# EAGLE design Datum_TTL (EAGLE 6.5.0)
dasdad

## Sheet 1 of 3: Tag
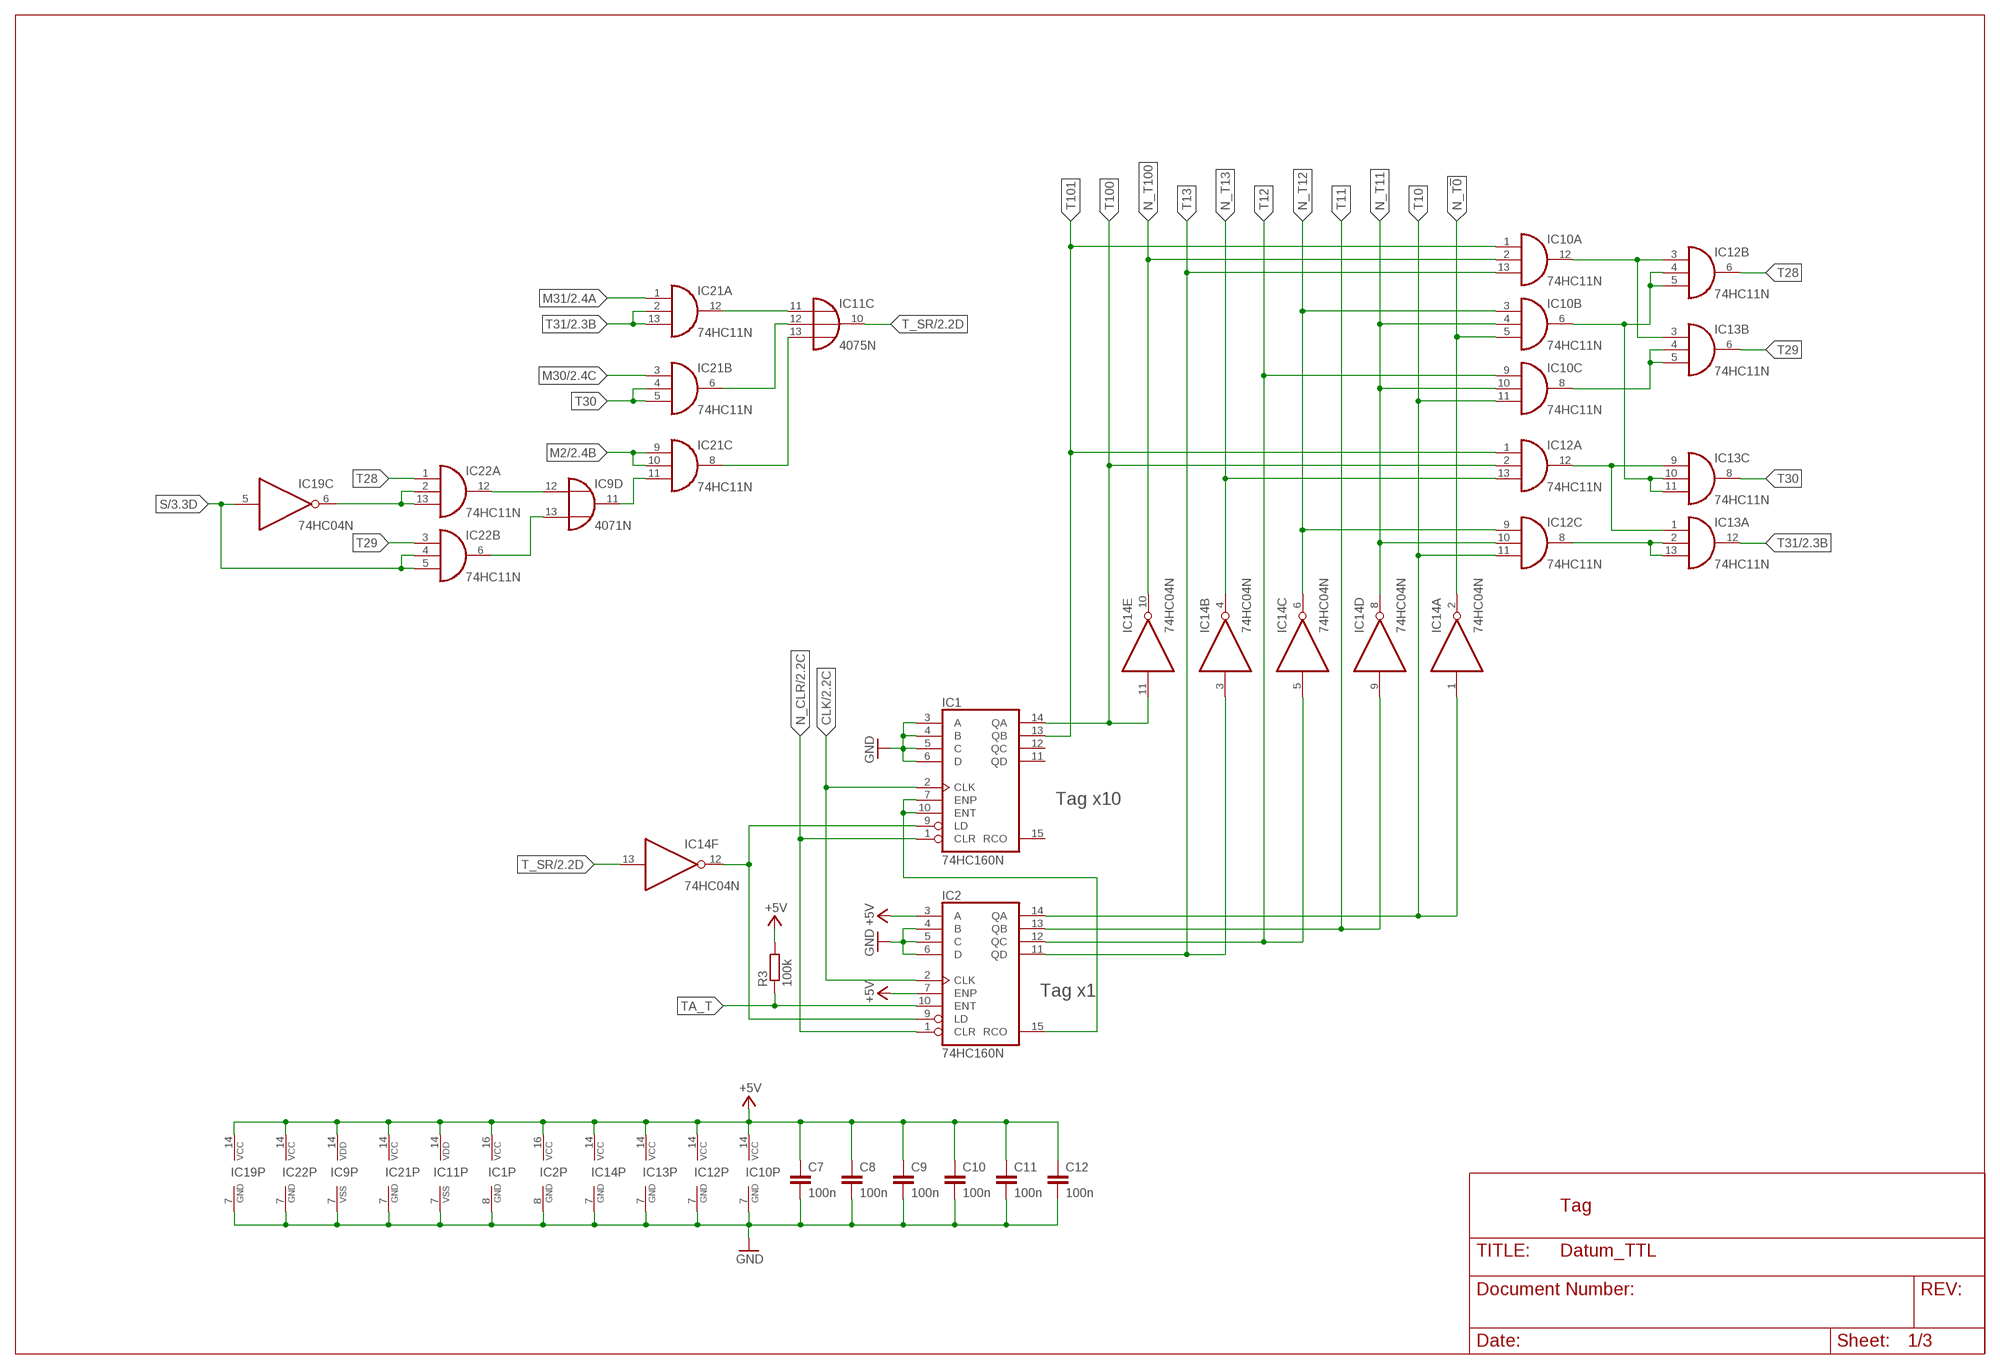
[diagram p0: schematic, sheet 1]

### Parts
C7  100n  C-EU025-024X044  [C025-024X044]
C8  100n  C-EU025-024X044  [C025-024X044]
C9  100n  C-EU025-024X044  [C025-024X044]
C10  100n  C-EU025-024X044  [C025-024X044]
C11  100n  C-EU025-024X044  [C025-024X044]
C12  100n  C-EU025-024X044  [C025-024X044]
IC1  74HC160N  [DIL16]
IC2  74HC160N  [DIL16]
IC9  4071N  [DIL14]
IC10  74HC11N  [DIL14]
IC11  4075N  [DIL14]
IC12  74HC11N  [DIL14]
IC13  74HC11N  [DIL14]
IC14  74HC04N  [DIL14]
IC19  74HC04N  [DIL14]
IC21  74HC11N  [DIL14]
IC22  74HC11N  [DIL14]
R3  100k  R-EU_0207/10  [0207/10]

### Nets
+5V: C7.1 C8.1 C9.1 C10.1 C11.1 C12.1 IC1.16(VCC) IC2.3(A) IC2.7(ENP) IC2.16(VCC) IC9.14(P:VDD) IC10.14(P:VCC) IC11.14(P:VDD) IC12.14(P:VCC) IC13.14(P:VCC) IC14.14(P:VCC) IC19.14(P:VCC) IC21.14(P:VCC) IC22.14(P:VCC) R3.2 ; also sheet 2,3
CLK: IC1.2(CLK) IC2.2(CLK) ; also sheet 2,3
GND: C7.2 C8.2 C9.2 C10.2 C11.2 C12.2 IC1.3(A) IC1.4(B) IC1.5(C) IC1.6(D) IC1.8(GND) IC2.4(B) IC2.5(C) IC2.6(D) IC2.8(GND) IC9.7(P:VSS) IC10.7(P:GND) IC11.7(P:VSS) IC12.7(P:GND) IC13.7(P:GND) IC14.7(P:GND) IC19.7(P:GND) IC21.7(P:GND) IC22.7(P:GND) ; also sheet 2,3
M2: IC21.9(C:I0) IC21.10(C:I1) ; also sheet 2
M30: IC21.3(B:I0) ; also sheet 2
M31: IC21.1(A:I0) ; also sheet 2
N$2: IC1.7(ENP) IC1.10(ENT) IC2.15(RCO)
N$21: IC10.12(A:O) IC12.3(B:I0) IC13.3(B:I0)
N$22: IC10.6(B:O) IC12.4(B:I1) IC12.5(B:I2) IC13.10(C:I1) IC13.11(C:I2)
N$23: IC12.8(C:O) IC13.2(A:I1) IC13.13(A:I2)
N$24: IC10.8(C:O) IC13.4(B:I1) IC13.5(B:I2)
N$25: IC12.12(A:O) IC13.1(A:I0) IC13.9(C:I0)
N$36: IC9.12(D:I0) IC22.12(A:O)
N$37: IC9.13(D:I1) IC22.6(B:O)
N$38: IC9.11(D:O) IC21.11(C:I2)
N$39: IC11.11(C:I0) IC21.12(A:O)
N$41: IC19.6(C:O) IC22.2(A:I1) IC22.13(A:I2)
N$42: IC11.12(C:I1) IC21.6(B:O)
N$43: IC11.13(C:I2) IC21.8(C:O)
N_CLR: IC1.1(CLR) IC2.1(CLR) ; also sheet 2,3
N_T11: IC10.4(B:I1) IC10.10(C:I1) IC12.10(C:I1) IC14.8(D:O)
N_T12: IC10.3(B:I0) IC12.9(C:I0) IC14.6(C:O)
N_T13: IC12.13(A:I2) IC14.4(B:O)
N_T100: IC10.2(A:I1) IC14.10(E:O)
N_T!0: IC10.5(B:I2) IC14.2(A:O)
N_T_SR: IC1.9(LD) IC2.9(LD) IC14.12(F:O)
S: IC19.5(C:I) IC22.4(B:I1) IC22.5(B:I2) ; also sheet 3
T10: IC2.14(QA) IC10.11(C:I2) IC12.11(C:I2) IC14.1(A:I) ; also sheet 3
T11: IC2.13(QB) IC14.9(D:I) ; also sheet 3
T12: IC2.12(QC) IC10.9(C:I0) IC14.5(C:I) ; also sheet 3
T13: IC2.11(QD) IC10.13(A:I2) IC14.3(B:I) ; also sheet 3
T28: IC12.6(B:O) IC22.1(A:I0)
T29: IC13.6(B:O) IC22.3(B:I0)
T30: IC13.8(C:O) IC21.4(B:I1) IC21.5(B:I2)
T31: IC13.12(A:O) IC21.2(A:I1) IC21.13(A:I2) ; also sheet 2
T100: IC1.14(QA) IC12.2(A:I1) IC14.11(E:I) ; also sheet 3
T101: IC1.13(QB) IC10.1(A:I0) IC12.1(A:I0) ; also sheet 3
T_SR: IC11.10(C:O) IC14.13(F:I) ; also sheet 2
TA_T: IC2.10(ENT) R3.1 ; also sheet 3
Unconnected: IC1.11(QD) IC1.12(QC) IC1.15(RCO)

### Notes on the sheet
- Tag x10
- Tag x1
- Tag

## Sheet 2 of 3: Monat
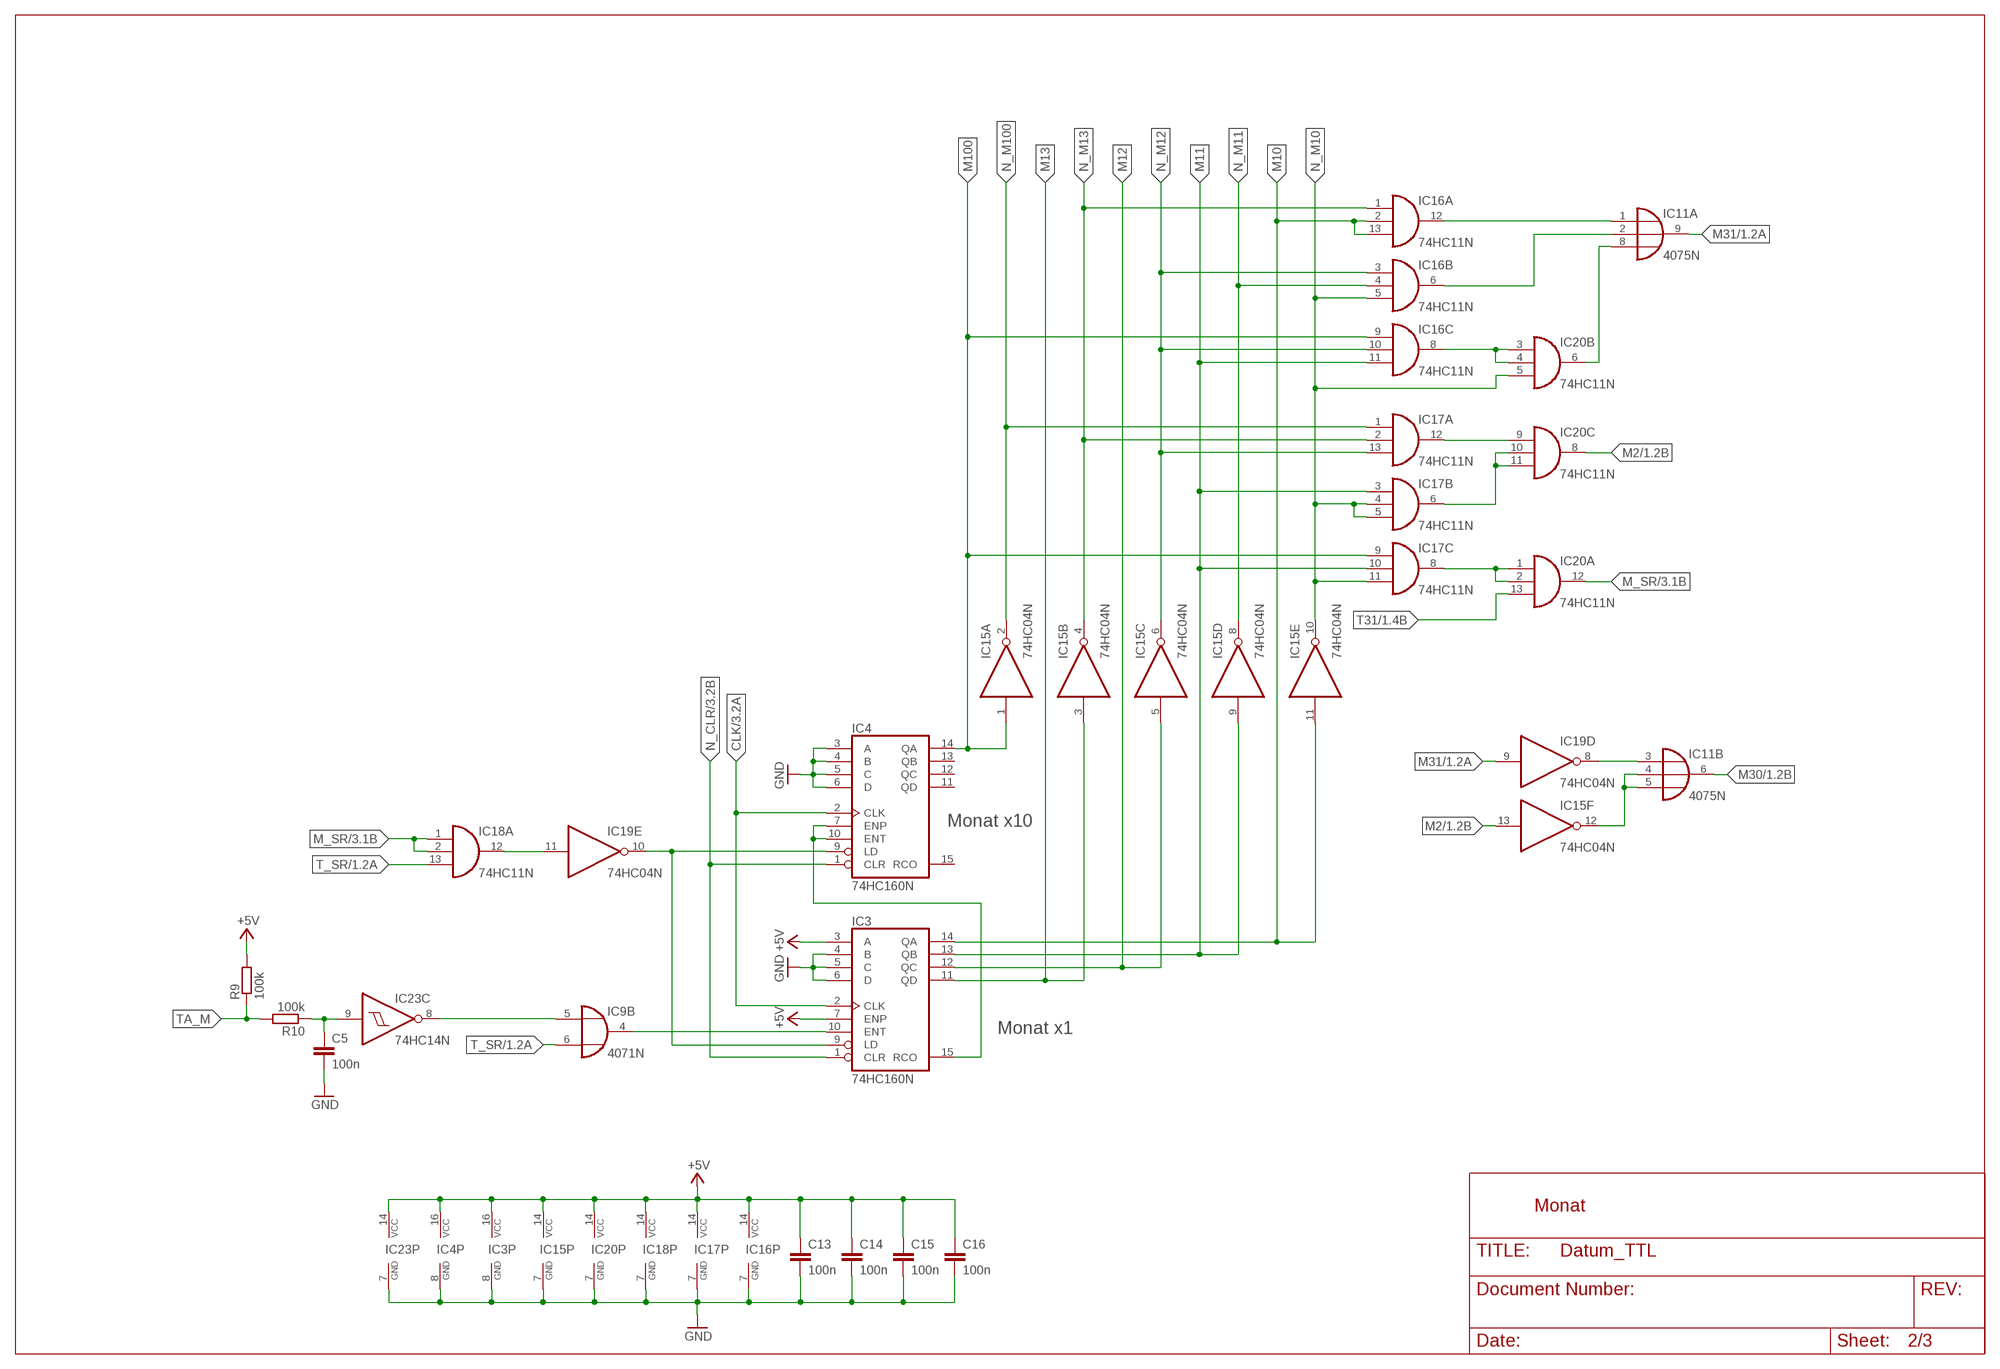
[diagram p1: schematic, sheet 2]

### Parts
C5  100n  C-EU025-024X044  [C025-024X044]
C13  100n  C-EU025-024X044  [C025-024X044]
C14  100n  C-EU025-024X044  [C025-024X044]
C15  100n  C-EU025-024X044  [C025-024X044]
C16  100n  C-EU025-024X044  [C025-024X044]
IC3  74HC160N  [DIL16]
IC4  74HC160N  [DIL16]
IC15  74HC04N  [DIL14]
IC16  74HC11N  [DIL14]
IC17  74HC11N  [DIL14]
IC18  74HC11N  [DIL14]
IC20  74HC11N  [DIL14]
IC23  74HC14N  [DIL14]
R9  100k  R-EU_0207/10  [0207/10]
R10  100k  R-EU_0207/10  [0207/10]

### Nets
+5V: C13.1 C14.1 C15.1 C16.1 IC3.3(A) IC3.7(ENP) IC3.16(VCC) IC4.16(VCC) IC15.14(P:VCC) IC16.14(P:VCC) IC17.14(P:VCC) IC18.14(P:VCC) IC20.14(P:VCC) IC23.14(P:VCC) R9.2 ; also sheet 1,3
CLK: IC3.2(CLK) IC4.2(CLK) ; also sheet 1,3
GND: C5.2 C13.2 C14.2 C15.2 C16.2 IC3.4(B) IC3.5(C) IC3.6(D) IC3.8(GND) IC4.3(A) IC4.4(B) IC4.5(C) IC4.6(D) IC4.8(GND) IC15.7(P:GND) IC16.7(P:GND) IC17.7(P:GND) IC18.7(P:GND) IC20.7(P:GND) IC23.7(P:GND) ; also sheet 1,3
M2: IC15.13(F:I) IC20.8(C:O) ; also sheet 1
M10: IC3.14(QA) IC15.11(E:I) IC16.2(A:I1) IC16.13(A:I2) ; also sheet 3
M11: IC3.13(QB) IC15.9(D:I) IC16.11(C:I2) IC17.3(B:I0) IC17.10(C:I1) ; also sheet 3
M12: IC3.12(QC) IC15.5(C:I) ; also sheet 3
M13: IC3.11(QD) IC15.3(B:I) ; also sheet 3
M30: IC11.6(B:O) ; also sheet 1
M31: IC11.9(A:O) IC19.9(D:I) ; also sheet 1
M100: IC4.14(QA) IC15.1(A:I) IC16.9(C:I0) IC17.9(C:I0) ; also sheet 3
M_SR: IC18.1(A:I0) IC18.2(A:I1) IC20.12(A:O) ; also sheet 3
N$3: IC9.5(B:I0) IC23.8(C:O)
N$4: IC18.12(A:O) IC19.11(E:I)
N$6: IC3.15(RCO) IC4.7(ENP) IC4.10(ENT)
N$7: IC3.10(ENT) IC9.4(B:O)
N$8: IC3.9(LD) IC4.9(LD) IC19.10(E:O)
N$14: IC17.8(C:O) IC20.1(A:I0) IC20.2(A:I1)
N$26: IC11.1(A:I0) IC16.12(A:O)
N$27: IC11.2(A:I1) IC16.6(B:O)
N$28: IC11.8(A:I2) IC20.6(B:O)
N$29: IC16.8(C:O) IC20.3(B:I0) IC20.4(B:I1)
N$30: IC17.12(A:O) IC20.9(C:I0)
N$31: IC17.6(B:O) IC20.10(C:I1) IC20.11(C:I2)
N$32: IC11.3(B:I0) IC19.8(D:O)
N$33: IC11.4(B:I1) IC11.5(B:I2) IC15.12(F:O)
N$77: C5.1 IC23.9(C:I) R10.1
N_CLR: IC3.1(CLR) IC4.1(CLR) ; also sheet 1,3
N_M10: IC15.10(E:O) IC16.5(B:I2) IC17.4(B:I1) IC17.5(B:I2) IC17.11(C:I2) IC20.5(B:I2)
N_M11: IC15.8(D:O) IC16.4(B:I1)
N_M12: IC15.6(C:O) IC16.3(B:I0) IC16.10(C:I1) IC17.13(A:I2)
N_M13: IC15.4(B:O) IC16.1(A:I0) IC17.2(A:I1)
N_M100: IC15.2(A:O) IC17.1(A:I0)
T31: IC20.13(A:I2) ; also sheet 1
T_SR: IC9.6(B:I1) IC18.13(A:I2) ; also sheet 1
TA_M: R9.1 R10.2 ; also sheet 3
Unconnected: IC4.11(QD) IC4.12(QC) IC4.13(QB) IC4.15(RCO)

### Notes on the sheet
- Monat x10
- Monat x1
- Monat

## Sheet 3 of 3: Jahr, Wochentag, IO
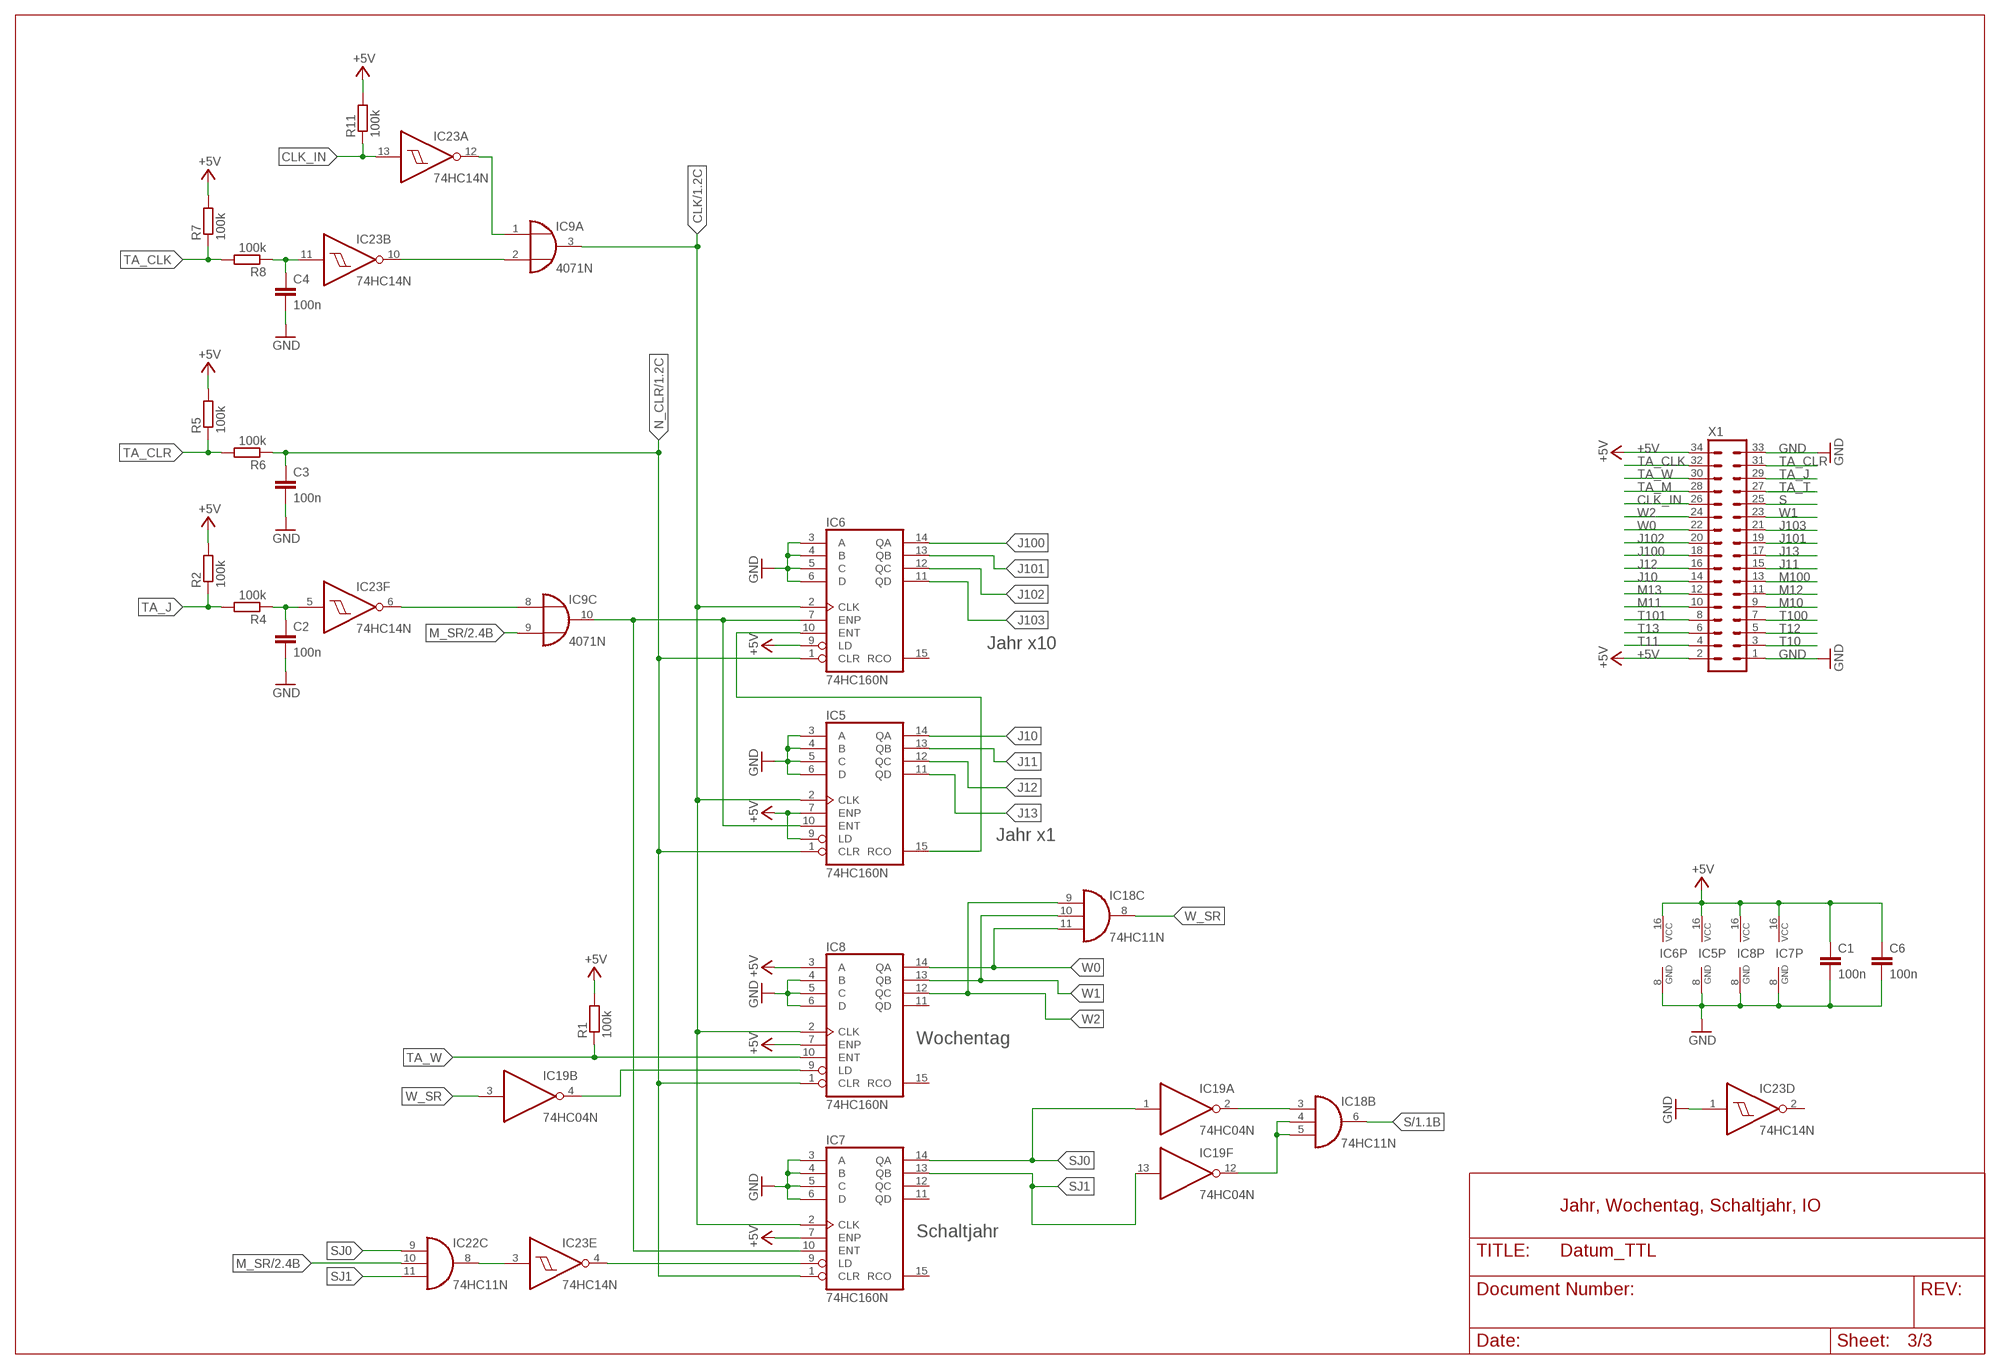
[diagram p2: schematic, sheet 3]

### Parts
C1  100n  C-EU025-024X044  [C025-024X044]
C2  100n  C-EU025-024X044  [C025-024X044]
C3  100n  C-EU025-024X044  [C025-024X044]
C4  100n  C-EU025-024X044  [C025-024X044]
C6  100n  C-EU025-024X044  [C025-024X044]
IC5  74HC160N  [DIL16]
IC6  74HC160N  [DIL16]
IC7  74HC160N  [DIL16]
IC8  74HC160N  [DIL16]
R1  100k  R-EU_0207/10  [0207/10]
R2  100k  R-EU_0207/10  [0207/10]
R4  100k  R-EU_0207/10  [0207/10]
R5  100k  R-EU_0207/10  [0207/10]
R6  100k  R-EU_0207/10  [0207/10]
R7  100k  R-EU_0207/10  [0207/10]
R8  100k  R-EU_0207/10  [0207/10]
R11  100k  R-EU_0207/10  [0207/10]
X1  ML34  [ML34]

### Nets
+5V: C1.1 C6.1 IC5.7(ENP) IC5.9(LD) IC5.16(VCC) IC6.9(LD) IC6.16(VCC) IC7.7(ENP) IC7.16(VCC) IC8.3(A) IC8.7(ENP) IC8.16(VCC) R1.2 R2.2 R5.2 R7.2 R11.2 X1.2 X1.34 ; also sheet 1,2
CLK: IC5.2(CLK) IC6.2(CLK) IC7.2(CLK) IC8.2(CLK) IC9.3(A:O) ; also sheet 1,2
CLK_IN: IC23.13(A:I) R11.1 X1.26
GND: C1.2 C2.2 C3.2 C4.2 C6.2 IC5.3(A) IC5.4(B) IC5.5(C) IC5.6(D) IC5.8(GND) IC6.3(A) IC6.4(B) IC6.5(C) IC6.6(D) IC6.8(GND) IC7.3(A) IC7.4(B) IC7.5(C) IC7.6(D) IC7.8(GND) IC8.4(B) IC8.5(C) IC8.6(D) IC8.8(GND) IC23.1(D:I) X1.1 X1.33 ; also sheet 1,2
J10: IC5.14(QA) X1.14
J11: IC5.13(QB) X1.15
J12: IC5.12(QC) X1.16
J13: IC5.11(QD) X1.17
J100: IC6.14(QA) X1.18
J101: IC6.13(QB) X1.19
J102: IC6.12(QC) X1.20
J103: IC6.11(QD) X1.21
M10: X1.9 ; also sheet 2
M11: X1.10 ; also sheet 2
M12: X1.11 ; also sheet 2
M13: X1.12 ; also sheet 2
M100: X1.13 ; also sheet 2
M_SR: IC9.9(C:I1) IC22.10(C:I1) ; also sheet 2
N$1: C2.1 IC23.5(F:I) R4.1
N$5: IC9.1(A:I0) IC23.12(A:O)
N$9: IC22.8(C:O) IC23.3(E:I)
N$10: IC5.15(RCO) IC6.10(ENT)
N$11: IC5.10(ENT) IC6.7(ENP) IC7.10(ENT) IC9.10(C:O)
N$13: IC7.9(LD) IC23.4(E:O)
N$15: IC9.8(C:I0) IC23.6(F:O)
N$16: IC8.9(LD) IC19.4(B:O)
N$17: IC9.2(A:I1) IC23.10(B:O)
N$19: C4.1 IC23.11(B:I) R8.1
N$34: IC18.3(B:I0) IC19.2(A:O)
N$35: IC18.4(B:I1) IC18.5(B:I2) IC19.12(F:O)
N_CLR: C3.1 IC5.1(CLR) IC6.1(CLR) IC7.1(CLR) IC8.1(CLR) R6.1 ; also sheet 1,2
S: IC18.6(B:O) X1.25 ; also sheet 1
SJ0: IC7.14(QA) IC19.1(A:I) IC22.9(C:I0)
SJ1: IC7.13(QB) IC19.13(F:I) IC22.11(C:I2)
T10: X1.3 ; also sheet 1
T11: X1.4 ; also sheet 1
T12: X1.5 ; also sheet 1
T13: X1.6 ; also sheet 1
T100: X1.7 ; also sheet 1
T101: X1.8 ; also sheet 1
TA_CLK: R7.1 R8.2 X1.32
TA_CLR: R5.1 R6.2 X1.31
TA_J: R2.1 R4.2 X1.29
TA_M: X1.28 ; also sheet 2
TA_T: X1.27 ; also sheet 1
TA_W: IC8.10(ENT) R1.1 X1.30
W0: IC8.14(QA) IC18.11(C:I2) X1.22
W1: IC8.13(QB) IC18.10(C:I1) X1.23
W2: IC8.12(QC) IC18.9(C:I0) X1.24
W_SR: IC18.8(C:O) IC19.3(B:I)
Unconnected: IC6.15(RCO) IC7.11(QD) IC7.12(QC) IC7.15(RCO) IC8.11(QD) IC8.15(RCO) IC23.2(D:O)

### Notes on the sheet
- Jahr x10
- Jahr x1
- Wochentag
- Jahr, Wochentag, Schaltjahr, IO
- Schaltjahr

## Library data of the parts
C1-C16 = rcl:C-EU: CAPACITOR, European symbol
IC1-IC8 = 74xx-eu:74*160: Synchronous 4-bit COUNTER
IC9 = 40xx:4071: Quad 2-input OR
IC10 IC12 IC13 IC16-IC18 IC20-IC22 = 74xx-eu:74*11: Triple 3-input AND gate
IC11 = 40xx:4075: Triple 3-input OR
IC14 IC15 IC19 = 74xx-eu:74*04: Hex INVERTER
IC23 = 74xx-eu:74*14: Hex schmitt trigger INVERTER
R1-R11 = rcl:R-EU_: RESISTOR, European symbol
X1 = con-harting-ml:ML34: HARTING; OC_FARNELL: unknown; OC_NEWARK: unknown

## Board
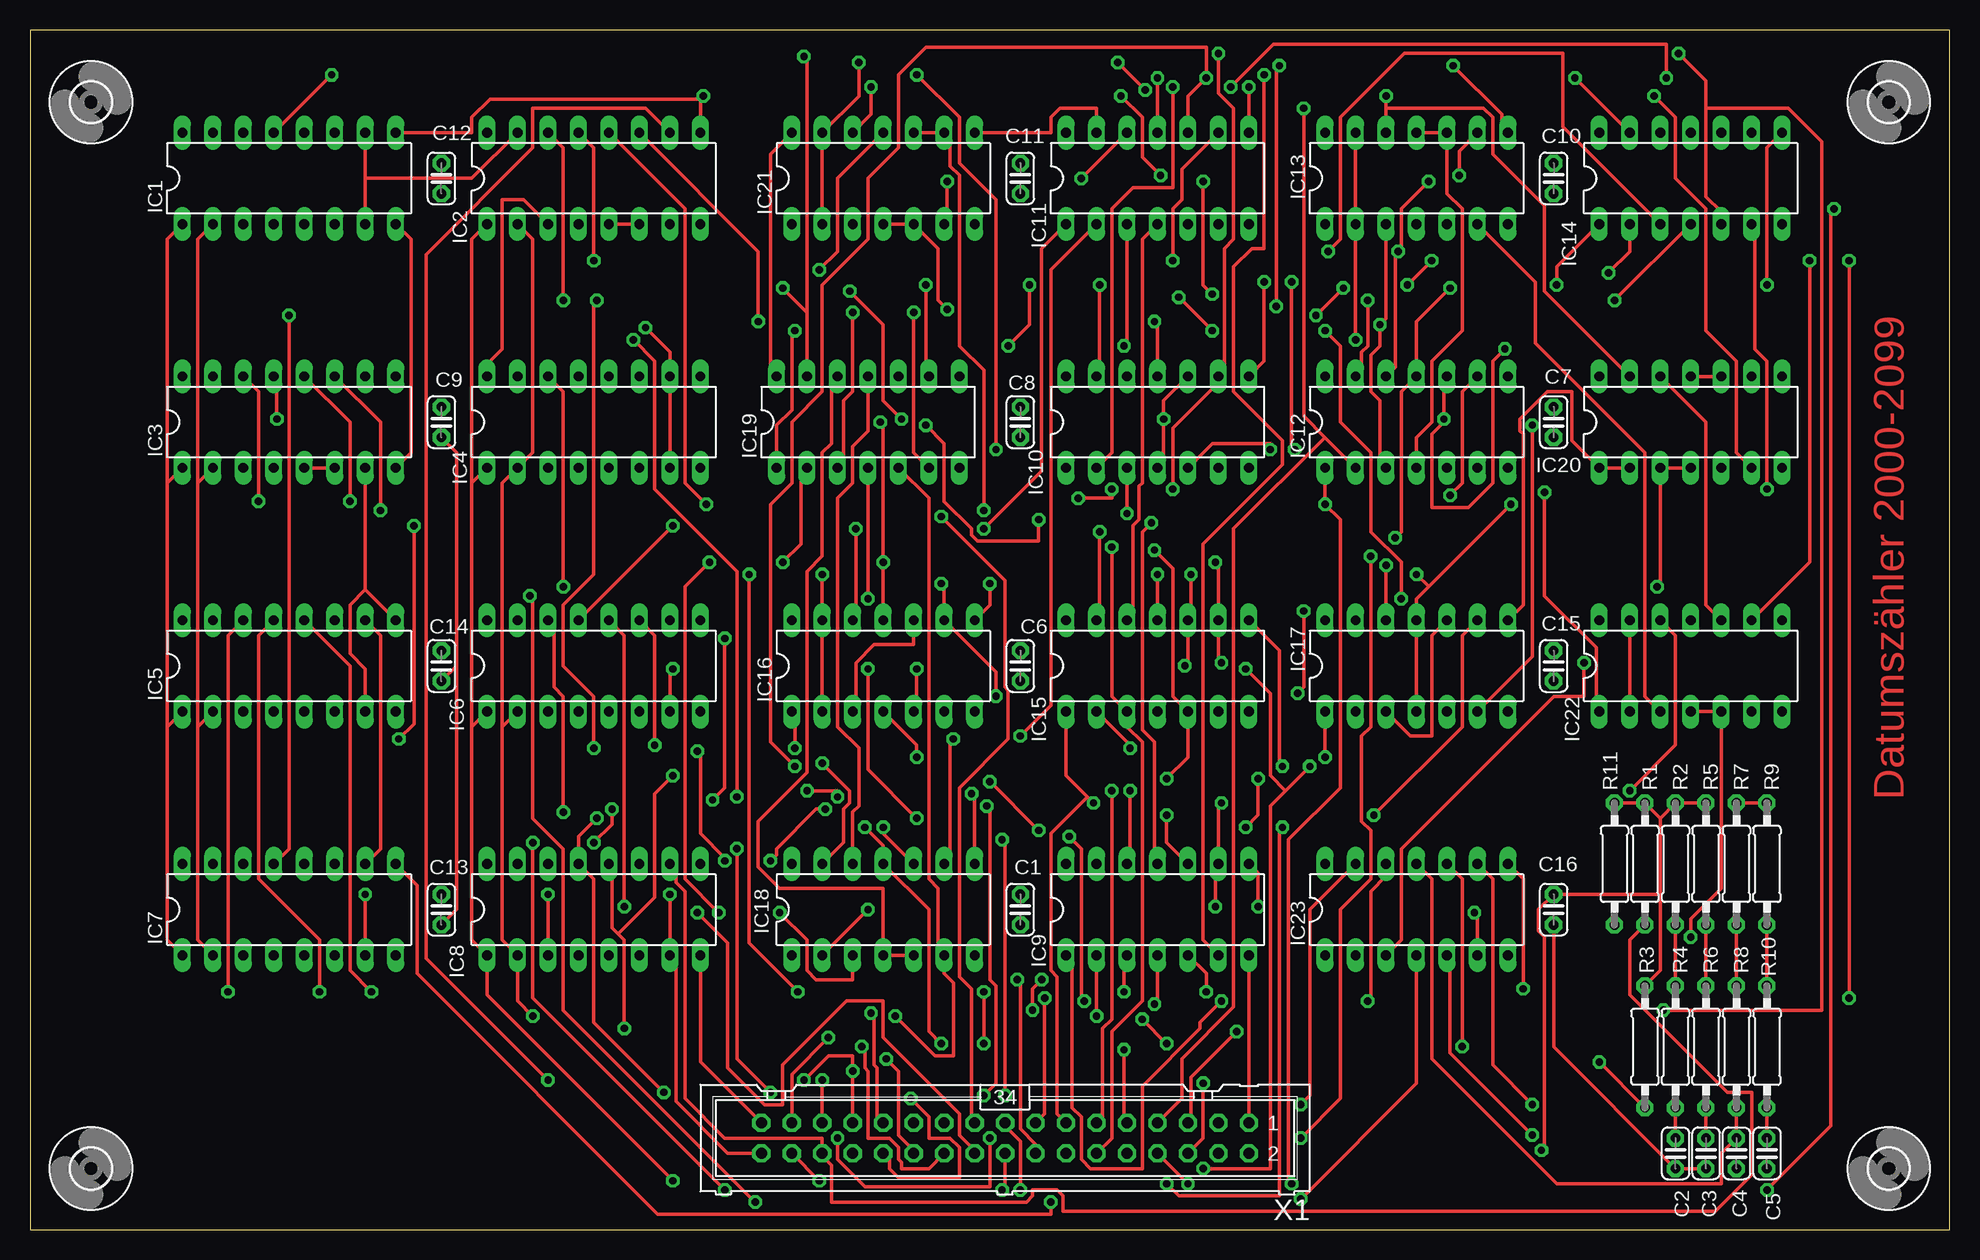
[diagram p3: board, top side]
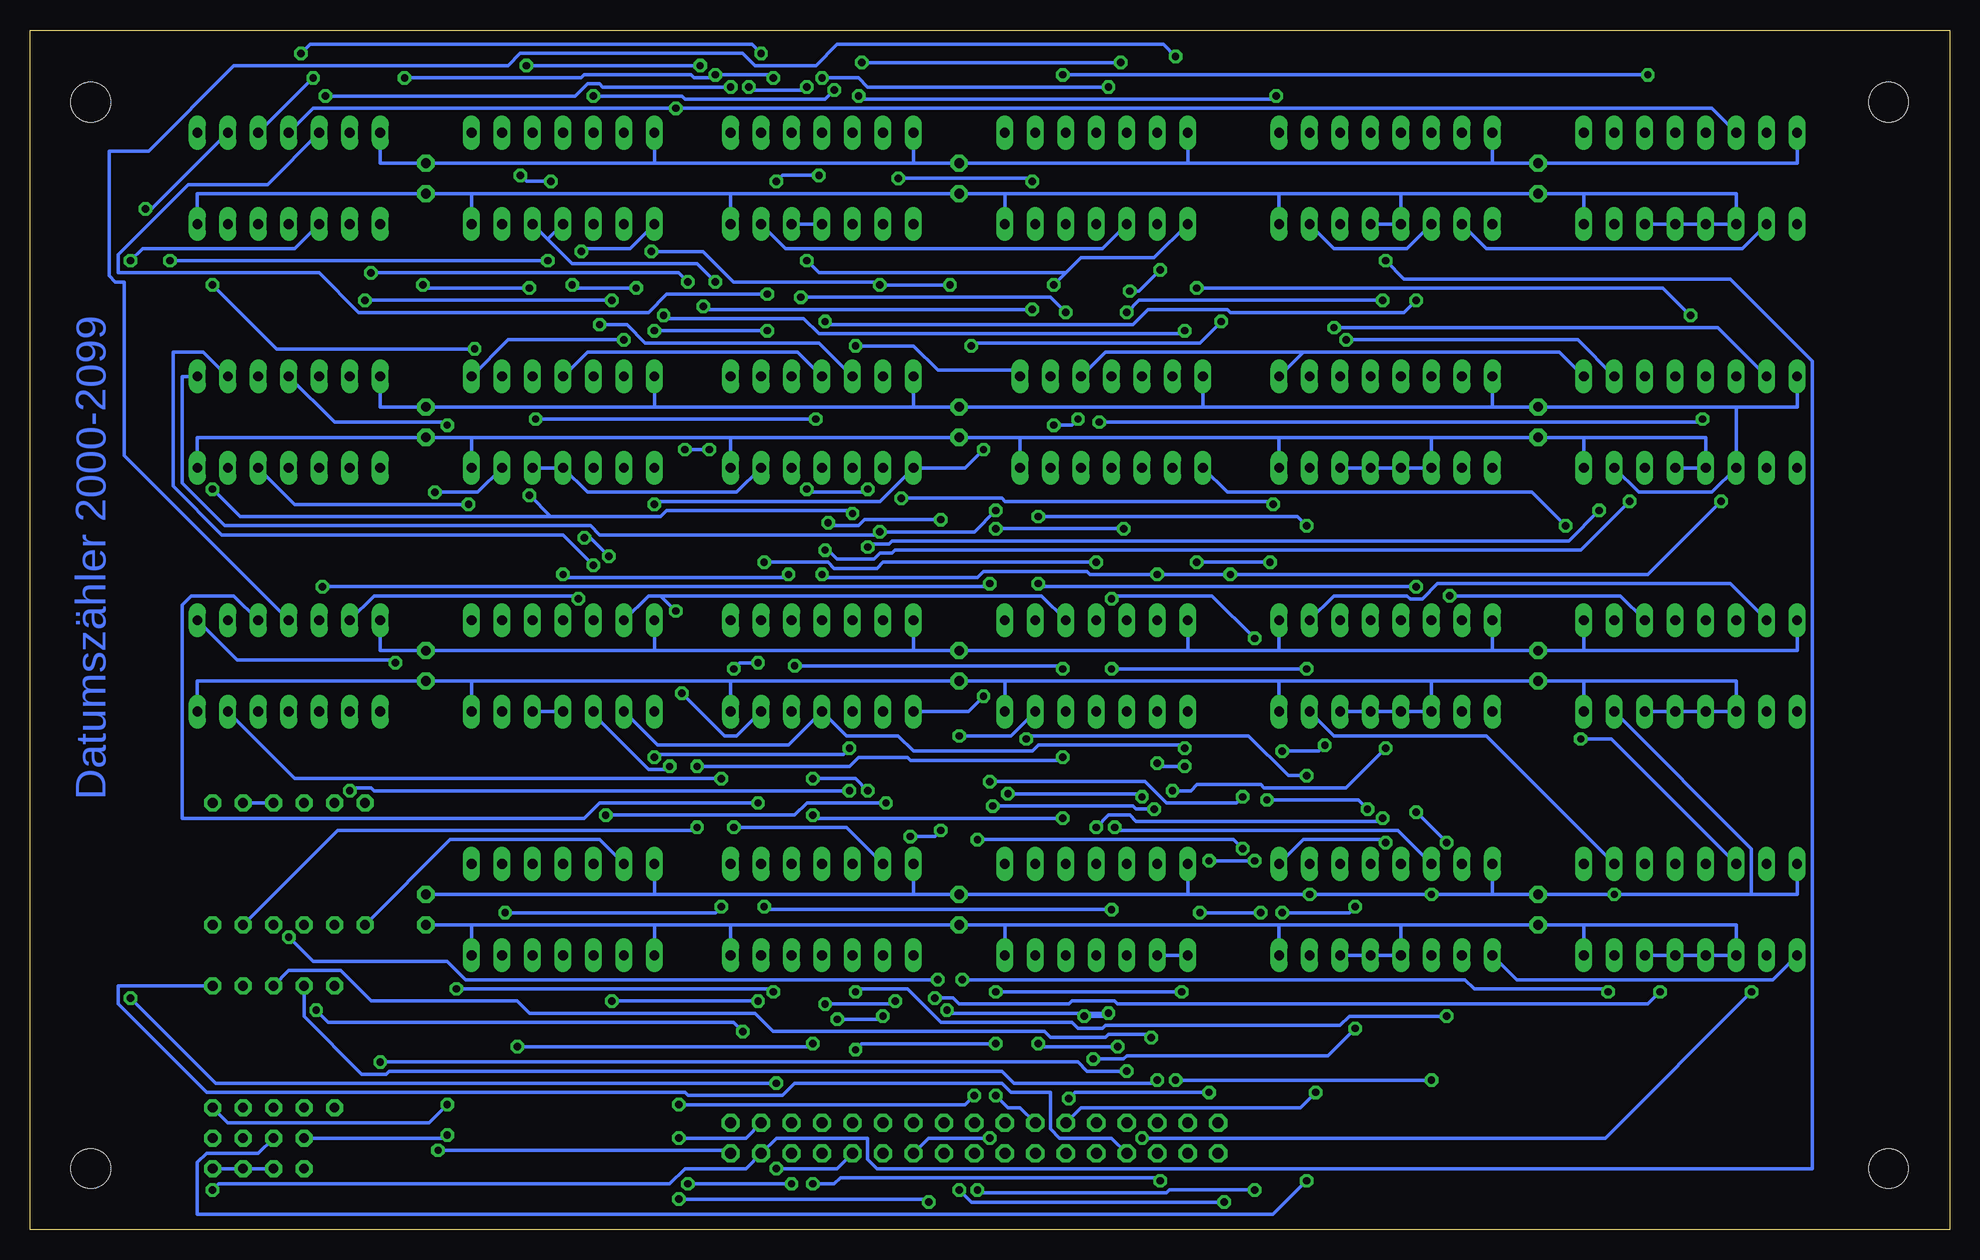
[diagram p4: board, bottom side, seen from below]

Size 160 x 100 mm. Coordinates in mm from the lower left corner, seen from the top.
Outline: 0,0 160,0 160,100 0,100 0,0
Copper layers (1*16): Top 0.035mm / dielectric 1.5mm / Bottom 0.035mm
Design rules "default *": minimum track width 12mil, minimum drill 24mil, track to track 12mil, track to pad 12mil, pad to pad 12mil, via to via 12mil, smd to smd 8mil, copper to edge 40mil, drill to drill 8mil, minimum pad ring 12mil, minimum via ring 10mil, stop-mask expansion 4mil, vias tented up to drill 0mil, thermal gap 10mil

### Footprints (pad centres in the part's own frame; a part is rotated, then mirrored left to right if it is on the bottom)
C025-024X044 = drill 0.813 octagon: 1 -1.27,0; 2 1.27,0
DIL16 = drill 0.813 long: 1 -8.89,-3.81; 2 -6.35,-3.81; 3 -3.81,-3.81; 4 -1.27,-3.81; 5 1.27,-3.81; 6 3.81,-3.81; 7 6.35,-3.81; 8 8.89,-3.81; 9 8.89,3.81; 10 6.35,3.81; 11 3.81,3.81; 12 1.27,3.81; 13 -1.27,3.81; 14 -3.81,3.81; 15 -6.35,3.81; 16 -8.89,3.81
DIL14 = drill 0.813 long: 1 -7.62,-3.81; 2 -5.08,-3.81; 3 -2.54,-3.81; 4 0,-3.81; 5 2.54,-3.81; 6 5.08,-3.81; 7 7.62,-3.81; 8 7.62,3.81; 9 5.08,3.81; 10 2.54,3.81; 11 0,3.81; 12 -2.54,3.81; 13 -5.08,3.81; 14 -7.62,3.81
0207/10 = drill 0.813 octagon: 1 -5.08,0; 2 5.08,0
3,3 = hole 3.3: 0,0
ML34 = drill 0.914 octagon: 1 -20.32,-1.27; 2 -20.32,1.27; 3 -17.78,-1.27; 4 -17.78,1.27; 5 -15.24,-1.27; 6 -15.24,1.27; 7 -12.7,-1.27; 8 -12.7,1.27; 9 -10.16,-1.27; 10 -10.16,1.27; 11 -7.62,-1.27; 12 -7.62,1.27; 13 -5.08,-1.27; 14 -5.08,1.27; 15 -2.54,-1.27; 16 -2.54,1.27; 17 0,-1.27; 18 0,1.27; 19 2.54,-1.27; 20 2.54,1.27; 21 5.08,-1.27; 22 5.08,1.27; 23 7.62,-1.27; 24 7.62,1.27; 25 10.16,-1.27; 26 10.16,1.27; 27 12.7,-1.27; 28 12.7,1.27; 29 15.24,-1.27; 30 15.24,1.27; 31 17.78,-1.27; 32 17.78,1.27; 33 20.32,-1.27; 34 20.32,1.27

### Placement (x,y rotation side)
C1  82.55,26.67 270 top
C2  137.16,6.35 270 top
C3  139.7,6.35 270 top
C4  142.24,6.35 270 top
C5  144.78,6.35 270 top
C6  82.55,46.99 270 top
C7  127,67.31 270 top
C8  82.55,67.31 270 top
C9  34.29,67.31 270 top
C10  127,87.63 270 top
C11  82.55,87.63 270 top
C12  34.29,87.63 270 top
C13  34.29,26.67 270 top
C14  34.29,46.99 270 top
C15  127,46.99 270 top
C16  127,26.67 270 top
IC1  21.59,87.63 0 top
IC2  46.99,87.63 0 top
IC3  21.59,67.31 0 top
IC4  46.99,67.31 0 top
IC5  21.59,46.99 0 top
IC6  46.99,46.99 0 top
IC7  21.59,26.67 0 top
IC8  46.99,26.67 0 top
IC9  93.98,26.67 0 top
IC10  93.98,67.31 0 top
IC11  93.98,87.63 0 top
IC12  115.57,67.31 0 top
IC13  115.57,87.63 0 top
IC14  138.43,87.63 0 top
IC15  93.98,46.99 0 top
IC16  71.12,46.99 0 top
IC17  115.57,46.99 0 top
IC18  71.12,26.67 0 top
IC19  69.85,67.31 0 top
IC20  138.43,67.31 0 top
IC21  71.12,87.63 0 top
IC22  138.43,46.99 0 top
IC23  115.57,26.67 0 top
R1  134.62,30.48 90 top
R2  137.16,30.48 90 top
R3  134.62,15.24 90 top
R4  137.16,15.24 90 top
R5  139.7,30.48 90 top
R6  139.7,15.24 90 top
R7  142.24,30.48 90 top
R8  142.24,15.24 90 top
R9  144.78,30.48 90 top
R10  144.78,15.24 90 top
R11  132.08,30.48 90 top
U$1  [3,3]  5.08,93.98 0 top
U$2  [3,3]  5.08,5.08 0 top
U$3  [3,3]  154.94,93.98 0 top
U$4  [3,3]  154.94,5.08 0 top
U$5  [A4L-LOC]  not placed on the board
X1  81.28,7.62 180 top

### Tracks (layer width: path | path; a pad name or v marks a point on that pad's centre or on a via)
+5V  (via drill 0.61)
  Top 0.305: IC2.3 41.15,85.85 39.37,85.85 39.37,73.41 38.1,72.14 IC4.16 | IC21.14 61.72,89.66 61.72,71.63 IC19.14 | 27.94,53.34 IC5.9 | IC3.7 27.94,53.34 | R9.2 R7.2 | R3.2 135.89,21.59 135.89,27.94 | 135.89,34.29 135.89,27.94 | 135.89,34.29 R1.2 R11.2 | 135.89,34.29 R2.2 R5.2 | X1.34 58.17,6.35 53.85,10.67 53.85,22.35 IC8.7 v53.34,27.94 | v27.94,27.94 IC7.7 | v43.18,27.94 IC8.3 | v125.98,6.6 126.24,6.86 126.24,24.38 125.73,24.89 125.73,26.67 C16.1 135.89,27.94 | 27.94,53.34 26.67,52.07 26.67,48.01 27.94,46.74 IC5.7
  Bottom 0.305: IC1.16 12.7,88.9 C12.1 38.1,88.9 | 38.1,88.9 63.5,88.9 | 63.5,88.9 C11.1 86.36,88.9 | 86.36,88.9 107.95,88.9 | 107.95,88.9 C10.1 130.81,88.9 IC14.14 | IC3.16 12.7,68.58 17.78,68.58 | 17.78,68.58 C9.1 38.1,68.58 | 38.1,68.58 62.23,68.58 | 62.23,68.58 C8.1 86.36,68.58 | 86.36,68.58 107.95,68.58 | 107.95,68.58 C7.1 130.81,68.58 IC20.14 | IC5.16 12.7,48.26 30.48,48.26 | 30.48,48.26 C14.1 38.1,48.26 | 38.1,48.26 55.88,48.26 | 55.88,48.26 63.5,48.26 | 63.5,48.26 C6.1 86.36,48.26 | 86.36,48.26 107.95,48.26 | 107.95,48.26 C15.1 130.81,48.26 IC22.14 | IC7.16 12.7,27.94 16.51,27.94 | 16.51,27.94 v27.94,27.94 C13.1 38.1,27.94 | 38.1,27.94 v43.18,27.94 v53.34,27.94 63.5,27.94 | 63.5,27.94 C1.1 86.36,27.94 | 86.36,27.94 107.95,27.94 | 107.95,27.94 C16.1 | IC8.16 38.1,27.94 | IC18.14 63.5,27.94 | IC9.14 86.36,27.94 | IC23.14 107.95,27.94 | IC15.14 86.36,48.26 | IC16.14 63.5,48.26 | IC17.14 107.95,48.26 | IC6.16 38.1,48.26 | IC4.16 38.1,68.58 | IC19.14 62.23,68.58 | IC10.14 86.36,68.58 | IC12.14 107.95,68.58 | IC13.14 107.95,88.9 | IC11.14 86.36,88.9 | IC21.14 63.5,88.9 | IC2.16 38.1,88.9 | 30.48,48.26 IC5.9 | 55.88,48.26 IC6.9 | IC2.3 45.21,81.79 51.31,81.79 IC2.7 | 17.78,68.58 IC3.3 19.81,61.47 25.91,61.47 IC3.7 | R5.2 R7.2 | IC5.7 16.51,31.75 16.51,27.94 | X1.2 101.85,6.6 v125.98,6.6
CLK  (via drill 0.61)
  Top 0.305: IC7.2 13.97,24.13 13.97,41.91 | IC5.2 13.97,41.91 | 13.97,62.23 IC3.2 | 13.97,41.91 13.97,62.23 | IC1.2 13.97,82.55 13.97,62.23 | 39.37,41.91 39.37,24.13 IC8.2 40.64,19.05 v41.91,17.78 | IC6.2 39.37,41.91 | IC9.3 91.19,22.61 v91.19,19.81 | 39.37,41.91 39.37,62.23 IC4.2 41.91,64.77 41.91,82.55 IC2.2
  Bottom 0.305: v91.19,19.81 90.93,20.07 86.87,20.07 84.07,17.27 73.15,17.27 72.64,16.76 70.61,16.76 70.36,17.02 50.8,17.02 50.04,17.78 v41.91,17.78 | IC1.2 17.27,81.79 38.61,81.79 IC2.2
CLK_IN  (via drill 0.61)
  Top 0.305: X1.26 71.63,5.84 71.63,5.08 72.39,4.32 77.47,4.32 77.47,6.86 76.71,7.62 74.93,7.62 74.93,9.4 v73.41,10.92 | v61.72,11.43 58.93,14.22 v58.93,31.75 | v81.03,32.51 81.28,32.26 v81.28,11.18 | v105.92,10.41 106.68,11.18 106.68,26.67 IC23.13
  Bottom 0.305: IC23.13 112.52,32.51 124.97,32.51 R11.1 | v73.41,10.92 72.9,11.43 v61.72,11.43 | v58.93,31.75 59.69,32.51 v81.03,32.51 | v81.28,11.18 82.04,10.41 v105.92,10.41
GND
  Top 0.305: C3.2 C2.2 127,15.24 C16.2 | X1.33 55.88,13.97 IC8.8 | IC9.7 X1.1 | IC2.6 IC2.5 | IC3.6 IC3.5 | 35.56,46.99 C14.2 | 35.56,46.99 35.56,64.77 C9.2 | IC1.8 31.75,82.55 31.75,64.77 IC3.8 | C13.2 35.56,26.67 35.56,46.99
  Bottom 0.305: 30.48,86.36 IC1.8 30.48,86.36 | 30.48,86.36 C12.2 45.72,86.36 | 45.72,86.36 55.88,86.36 | 55.88,86.36 78.74,86.36 | 78.74,86.36 C11.2 101.6,86.36 | 101.6,86.36 123.19,86.36 | 123.19,86.36 C10.2 146.05,86.36 IC14.7 | IC20.7 146.05,66.04 C7.2 123.19,66.04 | 123.19,66.04 101.6,66.04 | 101.6,66.04 C8.2 77.47,66.04 | 77.47,66.04 55.88,66.04 | 55.88,66.04 43.18,66.04 | 43.18,66.04 C9.2 30.48,66.04 | 30.48,66.04 20.32,66.04 IC3.4 IC3.5 | IC22.7 146.05,45.72 C15.2 123.19,45.72 | 123.19,45.72 101.6,45.72 | 101.6,45.72 C6.2 78.74,45.72 | 78.74,45.72 55.88,45.72 | 55.88,45.72 43.18,45.72 | 43.18,45.72 C14.2 30.48,45.72 | 30.48,45.72 17.78,45.72 IC5.3 IC5.4 IC5.5 IC5.6 | C16.2 123.19,25.4 | 123.19,25.4 107.95,25.4 | 107.95,25.4 101.6,25.4 | 101.6,25.4 C1.2 78.74,25.4 | 78.74,25.4 55.88,25.4 | 55.88,25.4 45.72,25.4 | 45.72,25.4 C13.2 30.48,25.4 | 30.48,25.4 17.78,25.4 IC7.3 19.05,22.86 IC7.4 IC7.5 IC7.6 | IC7.8 30.48,25.4 | 43.18,45.72 IC6.3 IC6.4 IC6.5 IC6.6 | IC16.7 78.74,45.72 | IC6.8 55.88,45.72 | IC5.8 30.48,45.72 | IC18.7 78.74,25.4 | IC8.8 55.88,25.4 | IC9.7 101.6,25.4 | IC23.7 123.19,25.4 | IC17.7 123.19,45.72 | IC15.7 101.6,45.72 | IC4.8 55.88,66.04 | IC19.7 77.47,66.04 | 43.18,66.04 IC4.3 IC4.4 IC4.5 IC4.6 | IC10.7 101.6,66.04 | IC12.7 123.19,66.04 | IC13.7 123.19,86.36 | IC11.7 101.6,86.36 | IC21.7 78.74,86.36 | IC2.8 55.88,86.36 | 30.48,86.36 17.78,86.36 IC1.3 IC1.4 IC1.5 IC1.6 | C3.2 C4.2 C5.2 | 45.72,25.4 IC8.4 IC8.5 IC8.6 | 107.95,25.4 IC23.1 | 45.72,86.36 IC2.4 IC2.5 | 30.48,66.04 IC3.8
J10  (via drill 0.61)
  Top 0.305: IC5.14 16.51,49.53 v16.51,19.81 | v67.31,7.62 67.31,5.84 69.6,3.56 80.01,3.56 v80.01,7.62
  Bottom 0.305: v16.51,19.81 28.7,7.62 v67.31,7.62 | v80.01,7.62 85.09,7.62 X1.14
J11  (via drill 0.61)
  Top 0.305: IC5.13 19.05,49.53 19.05,29.21 24.13,24.13 v24.13,19.81 | v84.58,19.3 84.58,9.65 X1.15
  Bottom 0.305: v24.13,19.81 25.15,18.8 69.34,18.8 69.6,19.05 73.15,19.05 73.41,18.8 82.55,18.8 83.06,19.3 v84.58,19.3
J12  (via drill 0.61)
  Top 0.305: IC5.12 26.67,46.99 26.67,21.59 v28.45,19.81 | v82.3,20.83 82.55,20.57 82.55,8.38 83.82,7.11 X1.16
  Bottom 0.305: v28.45,19.81 28.7,20.07 39.62,20.07 40.39,20.83 v82.3,20.83
J13  (via drill 0.61)
  Top 0.305: v41.66,52.83 41.91,52.58 41.91,34.29 44.45,31.75 44.45,18.29 v60.45,2.29 | v82.55,3.3 82.55,7.37 81.28,8.64 X1.17
  Bottom 0.305: IC5.11 27.43,52.83 v41.66,52.83 | v60.45,2.29 81.53,2.29 v82.55,3.3
J100  (via drill 0.61)
  Top 0.305: IC6.14 43.69,50.29 43.69,45.21 44.45,44.45 v44.45,34.8 | v41.91,32.26 41.91,19.3 v57.91,3.3 | v81.03,3.3 81.28,3.56 X1.18
  Bottom 0.305: v41.91,32.26 v44.45,34.8 | v57.91,3.3 65.02,3.3 65.28,3.05 80.77,3.05 v81.03,3.3
J101  (via drill 0.61)
  Top 0.305: v53.59,58.67 IC6.13 | v75.95,59.44 81.28,54.1 81.28,45.21 81.53,44.96 81.53,40.89 77.47,36.83 77.47,21.08 78.49,20.07 78.49,9.14 X1.19
  Bottom 0.305: v53.59,58.67 54.36,59.44 v75.95,59.44
J102  (via drill 0.61)
  Top 0.305: IC6.12 49.53,49.53 v49.53,26.92 | v55.63,26.42 58.17,23.88 58.17,13.46 61.21,10.41 62.74,10.41 62.74,13.72 68.07,19.05 71.12,19.05 71.12,16 77.47,9.65 77.47,7.87 78.74,6.6 X1.20
  Bottom 0.305: v49.53,26.92 50.04,26.42 v55.63,26.42
J103  (via drill 0.61)
  Top 0.305: IC6.11 52.07,49.53 v52.07,40.39 | v55.63,39.88 55.88,39.62 55.88,33.02 57.91,30.99 v57.91,30.73 | v61.72,30.73 62.23,31.24 62.23,31.75 65.53,35.05 v66.29,35.05 | v79.76,35.31 80.01,35.05 80.01,20.83 80.52,20.32 80.52,12.19 v79.5,11.18
  Bottom 0.305: v52.07,40.39 52.58,39.88 v55.63,39.88 | v61.72,30.73 v57.91,30.73 | v66.29,35.05 67.82,35.05 68.07,35.31 v79.76,35.31 | v79.5,11.18 78.49,10.16 77.47,10.16 X1.21
M2  (via drill 0.61)
  Top 0.305: IC21.10 IC21.9 76.71,90.93 76.71,88.65 77.47,87.88 77.47,73.66 79.5,71.63 v79.5,59.94 | IC15.13 89.15,51.05 v89.15,58.17
  Bottom 0.305: IC20.8 147.32,71.12 147.32,62.23 143.76,58.67 113.28,58.67 112.52,57.91 89.41,57.91 v89.15,58.17 81.28,58.17 v79.5,59.94
M10  (via drill 0.61)
  Top 0.305: IC16.2 IC16.13 v66.04,54.61 | IC3.14 19.05,69.85 v19.05,60.71 | v93.98,54.61 IC15.11 | X1.9 91.19,9.14 v91.19,14.99 | v79.5,19.81 v79.5,15.49 | v64.01,19.81 59.94,23.88 v59.94,54.61
  Bottom 0.305: v19.05,60.71 25.15,54.61 v59.94,54.61 v66.04,54.61 71.63,54.61 71.88,54.86 80.52,54.86 81.03,54.36 93.73,54.36 v93.98,54.61 | v91.19,14.99 90.68,15.49 v79.5,15.49 | v64.01,19.81 v79.5,19.81
M11  (via drill 0.61)
  Top 0.305: IC17.3 115.06,41.15 116.84,41.15 116.84,49.53 IC17.10 | v97.79,5.08 103.38,5.08 103.38,35.31 104.65,36.58 | v106.68,38.61 104.65,36.58 | IC16.11 v71.12,55.63 71.12,67.06 v70.87,67.31 | v98.81,55.63 99.06,55.37 IC15.9 99.06,47.5 v99.31,47.24 | IC3.13 20.57,70.87 v20.57,67.56 | 104.65,36.58 103.38,37.85 103.38,44.7 v101.35,46.74
  Bottom 0.305: X1.10 92.71,5.08 v97.79,5.08 | v106.68,38.61 106.93,38.35 108.46,38.35 113.03,42.93 IC17.3 | v71.12,55.63 88.9,55.63 89.41,55.12 92.96,55.12 93.47,55.63 v98.81,55.63 | v20.57,67.56 20.83,67.31 v70.87,67.31 | v101.35,46.74 100.84,47.24 v99.31,47.24
M12  (via drill 0.61)
  Top 0.305: IC3.12 26.67,67.31 v26.67,60.71 | v93.73,56.64 95.25,55.12 95.25,44.45 IC15.5 96.52,39.37 v94.74,37.59 | X1.11 89.41,9.4 89.41,16.76 90.17,17.53 v90.17,36.58
  Bottom 0.305: v26.67,60.71 30.73,56.64 87.88,56.64 88.14,56.39 89.15,56.39 89.66,55.88 92.71,55.88 93.47,56.64 v93.73,56.64 | v90.17,36.58 91.19,37.59 v94.74,37.59
M13  (via drill 0.61)
  Top 0.305: IC3.11 29.21,67.31 v29.21,59.94 | v90.17,56.9 90.17,44.45 IC15.3 91.44,41.91 92.71,40.64 92.71,19.05 90.17,16.51 90.17,7.62 X1.12
  Bottom 0.305: v29.21,59.94 31.75,57.4 88.14,57.4 88.39,57.15 89.92,57.15 v90.17,56.9
M30
  Bottom 0.305: IC21.3 70.61,81.79 97.03,81.79 IC11.6
M31  (via drill 0.61)
  Top 0.305: IC19.9 74.68,71.37 v74.68,78.74 | IC11.9 96.01,88.39 96.01,85.85 95.25,85.09 v95.25,80.77
  Bottom 0.305: 73.66,79.76 72.39,81.03 66.29,81.03 IC21.1 | 73.66,79.76 v74.68,78.74 | v95.25,80.77 94.23,79.76 73.66,79.76
M100  (via drill 0.61)
  Top 0.305: v80.52,44.45 80.52,46.48 IC16.9 76.2,53.59 v75.95,53.85 | IC17.9 119.38,49.53 119.38,41.91 v112.01,34.54 | 88.14,36.07 86.36,37.85 IC15.1 | 88.14,36.07 v88.65,35.56 | IC4.14 44.45,69.85 v44.45,53.59 | X1.13 85.6,9.65 85.6,21.08 85.09,21.59 85.09,33.02 88.14,36.07
  Bottom 0.305: v80.52,44.45 81.79,43.18 IC15.1 | v112.01,34.54 96.27,34.54 95.25,35.56 v88.65,35.56 | v44.45,53.59 75.69,53.59 v75.95,53.85
M_SR  (via drill 0.61)
  Top 0.305: IC22.10 139.7,52.07 139.7,67.31 IC20.12 | v98.81,26.92 98.81,30.23 IC9.9 99.06,35.31 v99.31,35.56 | IC18.2 v69.85,26.67
  Bottom 0.305: IC18.2 IC18.1 | v98.81,26.92 98.55,26.67 v69.85,26.67 | IC22.10 143,52.83 146.56,52.83 147.32,52.07 147.32,34.29 113.79,34.29 112.52,35.56 v99.31,35.56
N$1  (via drill 0.61)
  Top 0.305: R4.1 C2.1 | IC23.5 118.36,22.61 118.36,14.73 v125.22,7.87
  Bottom 0.305: v125.22,7.87 125.48,7.62 C2.1
N$2
  Top 0.305: IC1.10 27.94,87.63 | 27.94,87.63 IC1.7 | IC2.15 36.83,87.63 27.94,87.63
N$3  (via drill 0.61)
  Top 0.305: IC9.5 98.04,21.34 v98.04,19.81 | v124.46,20.07 124.46,29.21 IC23.8
  Bottom 0.305: v98.04,19.81 98.3,20.07 v124.46,20.07
N$4
  Top 0.305: IC18.12 68.58,34.8 69.09,35.31 69.09,40.13 67.31,41.91 67.31,60.96 68.58,62.23 68.58,65.28 69.85,66.55 IC19.11
N$5  (via drill 0.61)
  Top 0.305: IC9.1 86.87,22.35 86.87,10.16 87.63,9.4 87.63,5.84 88.39,5.08 92.71,5.08 92.71,11.94 97.54,16.76 97.54,17.27 v99.31,19.05 | v111.51,19.05 111.76,19.3 111.76,28.19 113.03,29.46 IC23.12
  Bottom 0.305: v111.51,19.05 v99.31,19.05
N$6  (via drill 0.61)
  Top 0.305: v51.31,75.18 53.34,73.15 IC4.10 IC4.7
  Bottom 0.305: IC3.15 19.3,75.18 v51.31,75.18
N$7  (via drill 0.61)
  Top 0.305: v50.29,74.17 52.07,72.39 52.07,61.72 58.93,54.86 v58.93,36.07 | v84.07,33.27 v80.01,37.34 | v86.61,32.77 87.63,31.75 87.63,19.3 v87.88,19.05 | v93.73,18.8 93.98,19.05 IC9.4
  Bottom 0.305: IC3.10 30.99,74.17 v50.29,74.17 | v58.93,36.07 59.44,35.56 65.28,35.56 67.06,37.34 v80.01,37.34 | v84.07,33.27 84.58,32.77 v86.61,32.77 | v87.88,19.05 88.14,18.8 v93.73,18.8
N$8
  Bottom 0.305: IC3.9 32.51,73.15 53.85,73.15 | IC4.9 53.85,73.15 | IC19.10 70.36,73.15 53.85,73.15
N$9  (via drill 0.61)
  Top 0.305: IC23.3 114.3,24.13 114.3,31.75 127,44.45 129.54,44.45 v129.54,47.24
  Bottom 0.305: v129.54,47.24 129.79,47.5 142.75,47.5 IC22.8
N$10
  Bottom 0.305: IC5.15 18.29,53.85 42.67,53.85 43.94,52.58 44.96,52.58 45.21,52.83 51.31,52.83 IC6.10
N$11  (via drill 0.61)
  Top 0.305: IC7.10 29.21,31.75 29.21,49.53 IC5.10 | IC9.10 94.74,32.26 v94.74,34.54 | v73.91,34.29 69.85,38.35 v69.85,46.74 | v53.59,46.74 53.34,46.48 IC6.7
  Bottom 0.305: IC6.7 51.31,41.15 38.61,41.15 IC7.10 | v94.74,34.54 94.49,34.29 v73.91,34.29 | v53.59,46.74 v69.85,46.74
N$13  (via drill 0.61)
  Top 0.305: IC7.9 32.26,28.7 32.26,21.34 52.32,1.27 85.09,1.27 v85.09,2.29 | v105.92,2.54 115.57,12.19 IC23.4
  Bottom 0.305: v85.09,2.29 85.34,2.54 v105.92,2.54
N$14
  Top 0.305: IC17.8 124.46,52.07 124.46,66.29 124.21,66.55 124.21,67.56 126.49,69.85 128.52,69.85 128.52,65.79 IC20.1 IC20.2
N$15  (via drill 0.61)
  Top 0.305: IC9.8 102.36,29.72 v102.36,26.92 | v120.4,26.42 120.65,26.16 IC23.6
  Bottom 0.305: v102.36,26.92 102.87,26.42 v120.4,26.42
N$16  (via drill 0.61)
  Top 0.305: v46.99,32.26 48.51,33.78 v48.51,35.05 | v56.9,35.81 57.91,36.83 v57.91,49.28 | IC19.4 v69.85,52.58
  Bottom 0.305: IC8.9 53.85,32.51 47.24,32.51 v46.99,32.26 | v48.51,35.05 49.28,35.81 v56.9,35.81 | v57.91,49.28 61.47,52.83 69.6,52.83 v69.85,52.58
N$17  (via drill 0.61)
  Top 0.305: v88.9,17.78 IC9.2 | v94.74,15.49 v92.71,17.53 | v119.38,15.24 119.38,29.21 IC23.10
  Bottom 0.305: v88.9,17.78 89.15,17.53 v92.71,17.53 | v94.74,15.49 95,15.24 v119.38,15.24
N$19
  Top 0.305: R8.1 C4.1 140.97,6.35 140.97,3.81 127.25,3.81 116.84,14.22 116.84,29.21 IC23.11
N$21  (via drill 0.61)
  Top 0.305: IC13.3 113.03,75.95 v112.52,75.44 112.52,73.66 111.76,72.9 111.76,69.85 112.52,69.09 112.52,64.01 IC12.3
  Bottom 0.305: IC10.12 94.23,73.91 108.71,73.91 110.24,75.44 v112.52,75.44
N$22
  Top 0.305: IC13.11 IC13.10 118.11,86.36 119.38,85.09 119.38,74.93 116.84,72.39 116.84,67.31 115.57,66.04 IC12.4
  Bottom 0.305: IC10.6 101.09,61.47 113.54,61.47 IC12.4 IC12.5
N$23  (via drill 0.61)
  Top 0.305: IC13.13 IC13.2 v110.49,74.17
  Bottom 0.305: IC12.8 120.14,74.17 v110.49,74.17
N$24  (via drill 0.61)
  Top 0.305: IC10.8 102.87,72.39 v102.87,78.99
  Bottom 0.305: v102.87,78.99 104.39,80.52 114.81,80.52 116.84,82.55 | IC13.5 116.84,82.55 | 116.84,82.55 IC13.4
N$25  (via drill 0.61)
  Top 0.305: IC12.12 113.79,71.88 113.79,81.28 v114.05,81.53 114.3,81.79 114.3,85.09 v116.59,87.38 | IC13.9 119.13,89.92 v119.13,87.88
  Bottom 0.305: v114.05,81.53 113.79,81.79 109.98,81.79 IC13.1 | v119.13,87.88 118.62,87.38 v116.59,87.38
N$26  (via drill 0.61)
  Top 0.305: IC16.12 68.83,51.05 v68.83,58.42 | v79.5,58.42 84.33,63.25 84.33,81.79 IC11.1
  Bottom 0.305: v79.5,58.42 v68.83,58.42
N$27  (via drill 0.61)
  Top 0.305: v82.55,41.15 85.09,43.69 85.09,80.01 IC11.2
  Bottom 0.305: IC16.6 78.23,41.15 v82.55,41.15
N$28  (via drill 0.61)
  Top 0.305: v101.6,95.25 IC11.8 | v135.38,94.49 137.16,92.71 137.16,87.63 139.7,85.09 139.7,74.93 142.24,72.39 142.24,64.77 IC20.6
  Bottom 0.305: v101.6,95.25 112.27,95.25 112.52,95.5 113.54,95.5 114.55,94.49 v135.38,94.49
N$29  (via drill 0.61)
  Top 0.305: IC16.8 80.01,52.07 v80.01,53.85 | v135.64,53.59 135.89,53.85 IC20.3 IC20.4
  Bottom 0.305: v80.01,53.85 80.26,53.59 v135.64,53.59
N$30  (via drill 0.61)
  Top 0.305: v113.03,55.37 IC17.12
  Bottom 0.305: v113.03,55.37 115.57,57.91 144.02,57.91 148.08,61.98 148.08,73.15 145.54,73.15 IC20.9
N$31  (via drill 0.61)
  Top 0.305: IC17.6 125.22,47.75 v125.22,67.06 | IC20.11 IC20.10
  Bottom 0.305: v125.22,67.06 125.48,67.31 134.62,67.31 IC20.11
N$32  (via drill 0.61)
  Top 0.305: v91.19,73.66 91.44,73.91 IC11.3
  Bottom 0.305: IC19.8 77.98,71.63 84.33,71.63 86.36,73.66 v91.19,73.66
N$33
  Top 0.305: IC15.12 91.95,51.31 91.95,58.67 92.46,59.18 92.46,61.98 92.71,62.23 92.71,82.55 IC11.4
  Bottom 0.305: IC11.4 IC11.5
N$34  (via drill 0.61)
  Top 0.305: IC19.2 64.26,62.99 64.26,57.15 v62.74,55.63 | v56.64,55.63 54.61,53.59 54.61,29.21 v57.4,26.42 | v62.48,26.42 64.77,24.13 64.77,21.59 65.53,20.83 68.58,20.83 IC18.3
  Bottom 0.305: v56.64,55.63 v62.74,55.63 | v62.48,26.42 v57.4,26.42
N$35
  Top 0.305: IC18.5 IC18.4 71.12,28.45 62.48,28.45 60.71,30.23 60.71,34.04 64.77,38.1 64.77,54.86 66.04,56.13 66.04,64.77 66.8,65.53 66.8,70.61 IC19.12
N$36  (via drill 0.61)
  Top 0.305: IC9.12 91.69,30.73 v91.69,36.58 | v133.35,36.58 137.16,40.39 137.16,49.53 IC22.12
  Bottom 0.305: v91.69,36.58 131.32,36.58 131.57,36.83 133.1,36.83 v133.35,36.58
N$37  (via drill 0.61)
  Top 0.305: v101.35,33.53 102.36,34.54 v102.36,37.59
  Bottom 0.305: IC9.13 91.95,33.53 v101.35,33.53 | v102.36,37.59 137.92,37.59 IC22.6
N$38  (via drill 0.61)
  Top 0.305: IC21.11 67.31,87.63 67.31,81.53 v65.79,80.01 | v68.33,78.23 71.12,75.44 71.12,69.09 v72.64,67.56 | v74.68,67.06 76.2,65.53 76.2,60.71 78.49,58.42 78.49,57.91 78.99,57.4 84.07,57.4 v84.07,59.18 | v93.47,58.93 92.71,58.17 92.71,41.66 93.73,40.64 93.73,30.73 IC9.11
  Bottom 0.305: v65.79,80.01 67.56,78.23 v68.33,78.23 | v72.64,67.56 73.15,67.06 v74.68,67.06 | v84.07,59.18 90.42,59.18 90.93,58.67 93.22,58.67 v93.47,58.93
N$39  (via drill 0.61)
  Top 0.305: IC21.12 70.1,92.96 v70.1,95.25 | IC11.11 v93.98,96.01
  Bottom 0.305: v70.1,95.25 90.17,95.25 90.93,96.01 v93.98,96.01
N$41  (via drill 0.61)
  Top 0.305: IC22.13 IC22.2 | IC19.6 73.66,64.77 v73.66,76.45 | v98.55,74.93 v95.76,77.72 | v107.95,74.93 109.22,73.66 109.22,67.31 111.76,64.77 111.76,58.17 114.3,55.63 v114.3,52.58
  Bottom 0.305: v73.66,76.45 74.93,77.72 v95.76,77.72 | v107.95,74.93 v98.55,74.93 | v114.3,52.58 114.55,52.83 131.32,52.83 IC22.13
N$42  (via drill 0.61)
  Top 0.305: IC21.6 76.45,84.07 v76.45,87.38 | IC11.12 v87.63,87.63
  Bottom 0.305: v76.45,87.38 76.71,87.63 v87.63,87.63
N$43
  Top 0.305: IC21.8 85.09,91.44 85.09,92.71 85.85,93.47 88.9,93.47 IC11.13
N$77  (via drill 0.61)
  Top 0.305: R10.1 C5.1 | IC23.9 121.92,29.21 121.92,13.72 v125.22,10.41
  Bottom 0.305: v125.22,10.41 126.75,8.89 143.51,8.89 R10.1
N_CLR  (via drill 0.61)
  Top 0.305: IC7.1 11.43,24.13 11.43,41.91 | IC5.1 11.43,41.91 | 11.43,62.23 IC3.1 | 11.43,41.91 11.43,62.23 | IC1.1 11.43,82.55 11.43,62.23 | R6.1 C3.1 | 36.83,41.91 36.83,24.13 IC8.1 38.1,19.56 v53.59,4.06 | IC6.1 36.83,41.91 | 36.83,62.23 IC4.1 | 36.83,41.91 36.83,62.23 | IC2.1 36.83,82.55 36.83,62.23
  Bottom 0.305: C3.1 140.97,6.35 145.29,6.35 146.05,5.59 146.05,1.27 56.39,1.27 v53.59,4.06 | IC7.1 14.73,20.83 36.07,20.83 IC8.1
N_M10  (via drill 0.61)
  Top 0.305: IC16.5 73.91,43.43 v73.91,46.74 | v96.27,46.99 96.52,47.24 IC15.10 96.77,51.05 v96.77,54.61 | IC17.4 IC17.11 115.57,52.58 116.59,53.59 | 116.59,53.59 v123.44,60.45 | 116.59,53.59 v115.57,54.61
  Bottom 0.305: v73.91,46.74 74.17,46.99 v96.27,46.99 | IC17.5 IC17.4 | IC20.5 137.92,60.45 v123.44,60.45 | v96.77,54.61 97.03,54.36 115.32,54.36 v115.57,54.61
N_M11  (via drill 0.61)
  Top 0.305: IC16.4 73.91,40.39 v73.91,39.37 | v104.39,38.61 104.14,38.86 104.14,48.26 IC15.8
  Bottom 0.305: v73.91,39.37 74.17,39.12 86.61,39.12 86.87,39.37 90.93,39.37 91.69,38.61 v104.39,38.61
N_M12  (via drill 0.61)
  Top 0.305: IC16.3 68.83,43.43 68.83,47.24 70.36,48.77 73.66,48.77 IC16.10 | v105.66,44.7 106.17,45.21 v106.17,51.56
  Bottom 0.305: IC15.6 101.09,41.15 102.11,41.15 v105.66,44.7 | 107.44,52.83 v106.17,51.56 | 107.44,52.83 108.46,52.83 IC17.13 | IC16.10 75.69,52.83 107.44,52.83
N_M13  (via drill 0.61)
  Top 0.305: IC16.1 63.75,42.93 v63.75,40.13
  Bottom 0.305: v63.75,40.13 64.01,40.39 75.95,40.39 76.45,39.88 86.36,39.88 87.63,41.15 91.95,41.15 IC15.4 96.77,40.39 107.7,40.39 IC17.2
N_M100  (via drill 0.61)
  Top 0.305: IC15.2 91.69,40.39 v91.69,40.13 | IC17.1 v107.95,39.37
  Bottom 0.305: v91.69,40.13 92.2,39.62 107.7,39.62 v107.95,39.37
N_T11  (via drill 0.61)
  Top 0.305: IC10.4 94.49,64.01 v94.49,67.56 94.49,69.09 IC10.10 | IC12.10 117.86,70.87 v117.86,67.56 117.86,67.31 116.84,66.29 116.84,60.2 119.89,60.2 121.92,62.23 121.92,72.39 v122.94,73.41 | IC14.8 144.78,90.17 v144.78,78.74
  Bottom 0.305: v94.49,67.56 v117.86,67.56 | v144.78,78.74 139.45,73.41 v122.94,73.41
N_T12  (via drill 0.61)
  Top 0.305: v91.44,59.69 IC10.3 | v118.36,61.21 119.38,62.23 119.38,69.85 IC12.9 | IC14.6 143.76,83.57 143.76,73.41 144.78,72.39 v144.78,61.72
  Bottom 0.305: v91.44,59.69 91.69,59.94 106.93,59.94 107.44,59.44 116.59,59.44 | v118.36,61.21 116.59,59.44 | v144.78,61.72 142.49,59.44 116.59,59.44
N_T13  (via drill 0.61)
  Top 0.305: IC12.13 111,71.63 111,73.15 111.51,73.66 v111.51,77.47 | IC14.4 v132.08,77.47
  Bottom 0.305: v132.08,77.47 v111.51,77.47
N_T100  (via drill 0.61)
  Top 0.305: IC10.2 90.17,64.77 90.17,85.09 91.95,86.87 95.25,86.87 v95.25,95.25 | v100.08,95.25 103.63,98.81 136.4,98.81 v136.4,96.01
  Bottom 0.305: v95.25,95.25 95.5,95 99.82,95 v100.08,95.25 | IC14.10 v136.4,96.01
N_T!0  (via drill 0.61)
  Top 0.305: IC10.5 98.55,65.53 103.38,65.53 v103.38,65.02 | v105.41,65.02 105.16,65.28 v105.16,78.99 | v131.57,79.76 133.35,81.53 IC14.2
  Bottom 0.305: v105.41,65.02 v103.38,65.02 | v105.16,78.99 105.92,79.76 v131.57,79.76
N_T_SR  (via drill 0.61)
  Top 0.305: IC1.9 36.83,91.44 36.83,92.71 38.35,94.23 55.88,94.23 | IC2.9 55.88,94.23 | v98.55,77.98 97.79,78.74 v97.79,87.38 | v94.23,87.88 92.71,89.41 92.71,92.71 v90.93,94.49 | 55.88,94.23 v56.13,94.49
  Bottom 0.305: IC14.12 140.21,87.12 146.81,87.12 152.65,81.28 152.65,79.76 135.89,79.76 132.59,76.45 108.46,76.45 106.93,77.98 v98.55,77.98 | v97.79,87.38 97.28,87.88 v94.23,87.88 | v90.93,94.49 90.68,94.23 56.39,94.23 v56.13,94.49
S  (via drill 0.61)
  Top 0.305: IC22.4 IC22.5 140.97,28.45 138.43,25.91 v138.43,24.38 | IC19.5 74.93,60.96 74.93,29.21 75.69,28.45 75.69,23.37 IC18.6 76.2,21.34 76.96,20.57 76.96,14.48 75.44,14.48 v72.14,17.78 | X1.25 70.61,9.4 70.61,13.46 70.36,13.72 70.36,17.78 v70.1,18.03 | v84.33,20.83 83.57,20.07 v83.57,18.29
  Bottom 0.305: v72.14,17.78 70.36,17.78 v70.1,18.03 83.31,18.03 v83.57,18.29 | v138.43,24.38 136.4,22.35 125.22,22.35 123.7,20.83 v84.33,20.83
SJ0  (via drill 0.61)
  Top 0.305: v30.73,40.89 32,42.16 v32,58.67 | IC22.9 148.34,55.63 v148.34,80.77 | v114.81,78.74 v116.84,80.77 | v107.19,76.2 v109.47,78.49 | v63.75,74.93 63.5,74.68 63.5,68.33 62.23,67.06 IC19.1
  Bottom 0.305: IC7.14 28.19,40.89 v30.73,40.89 | v32,58.67 34.8,61.47 60.2,61.47 IC19.1 | v116.84,80.77 v148.34,80.77 | v114.81,78.74 114.55,78.49 v109.47,78.49 | v107.19,76.2 106.93,75.95 95.5,75.95 94.23,74.68 64.01,74.68 v63.75,74.93
SJ1  (via drill 0.61)
  Top 0.305: IC7.13 21.59,31.75 v21.59,76.2 | 64.77,76.45 v62.74,78.49 | IC19.13 64.77,76.45 | v64.52,97.79 64.77,97.54 64.77,76.45
  Bottom 0.305: v21.59,76.2 23.88,78.49 v62.74,78.49 | IC22.11 152.15,64.52 152.15,78.99 152.91,78.99 153.42,79.5 153.42,89.92 150.11,89.92 143,97.03 120.14,97.03 119.13,98.04 100.58,98.04 99.57,97.03 94.49,97.03 92.71,98.81 65.53,98.81 v64.52,97.79
T10  (via drill 0.61)
  Top 0.305: IC14.1 127.25,80.26 v127.25,78.74 | v118.36,78.49 115.57,75.69 IC12.11 114.3,69.85 114.3,58.17 v113.79,57.66 | IC2.14 44.45,90.17 v44.45,77.47 | v93.73,75.69 93.98,75.44 IC10.11 | v105.92,7.62 109.22,10.92 109.22,26.67 111.76,29.21 111.76,33.27 111,34.04 111,41.15 111.76,41.91 v111.76,56.13
  Bottom 0.305: IC10.11 96.01,73.15 113.54,73.15 IC12.11 | v127.25,78.74 127,78.49 v118.36,78.49 | v44.45,77.47 45.47,76.45 59.94,76.45 60.2,76.71 66.8,76.71 68.07,75.44 93.47,75.44 v93.73,75.69 | X1.3 100.33,7.62 v105.92,7.62 | v111.76,56.13 113.28,57.66 v113.79,57.66
T11  (via drill 0.61)
  Top 0.305: IC2.13 46.99,90.17 v46.99,80.77 | v150.37,85.09 150.11,84.84 150.11,8.64 v144.78,3.3
  Bottom 0.305: v46.99,80.77 45.47,79.25 18.29,79.25 11.43,72.39 11.43,5.08 89.41,5.08 90.17,5.84 90.17,7.62 97.79,7.62 X1.4 100.33,5.08 105.41,5.08 106.68,3.81 144.27,3.81 v144.78,3.3 | IC14.9 149.86,85.09 v150.37,85.09
T12  (via drill 0.61)
  Top 0.305: v99.06,98.04 99.06,94.74 100.33,93.47 100.33,82.55 99.57,81.79 99.57,71.63 IC10.9 99.06,70.61 95.25,66.8 v95.25,61.72 | v137.41,98.04 139.7,95.76 139.7,93.47 | 139.7,93.47 139.7,86.11 140.97,84.84 IC14.5 | IC2.12 54.61,85.09 54.61,62.23 v56.39,60.45 | v87.38,60.96 90.17,60.96 v90.17,61.72 | X1.5 96.77,9.14 96.77,12.7 v100.58,16.51 | v136.14,18.29 149.35,18.29 149.35,90.68 146.56,93.47 139.7,93.47
  Bottom 0.305: v99.06,98.04 99.82,98.81 136.65,98.81 v137.41,98.04 | v56.39,60.45 56.64,60.71 78.74,60.71 78.99,60.96 v87.38,60.96 | v90.17,61.72 90.42,61.47 95,61.47 v95.25,61.72 | v100.58,16.51 101.35,17.27 135.13,17.27 v136.14,18.29
T13  (via drill 0.61)
  Top 0.305: IC10.13 89.15,71.37 v89.15,78.74 | v108.2,81.53 109.22,82.55 109.22,92.71 114.55,98.04 127.76,98.04 127.76,91.95 IC14.3 | IC2.11 60.71,81.53 v60.71,75.69 | v81.53,73.66 83.31,75.44 v83.31,78.74 | X1.6 97.79,7.62 v97.79,12.19 | v151.64,80.77 v151.64,19.3
  Bottom 0.305: v108.2,81.53 103.89,81.53 101.35,78.99 89.41,78.99 v89.15,78.74 v83.31,78.74 | v60.71,75.69 62.48,73.91 81.28,73.91 v81.53,73.66 | v97.79,12.19 144.53,12.19 v151.64,19.3 | v151.64,80.77 150.62,81.79 137.92,81.79 IC14.3
T28  (via drill 0.61)
  Top 0.305: IC22.1 130.56,43.43 130.56,48.51 126.24,52.83 v126.24,61.47
  Bottom 0.305: v126.24,61.47 122.68,61.47 IC12.6
T29
  Top 0.305: IC22.3 134.62,44.45 134.62,64.77 125.48,73.91 125.48,78.99 IC13.6
T30  (via drill 0.61)
  Top 0.305: IC21.4 IC21.5 75.69,81.79 75.69,77.47 v76.45,76.71 | IC13.8 122.68,91.95 122.68,92.96 v118.62,97.03 | v104.14,97.03 103.89,96.77 v103.89,76.96
  Bottom 0.305: v104.14,97.03 v118.62,97.03 | v103.89,76.96 103.63,76.71 v76.45,76.71
T31  (via drill 0.61)
  Top 0.305: IC21.2 IC21.13 69.09,94.49 v69.09,97.28 | IC20.13 126.24,78.23 126.24,85.34 121.92,89.66 121.92,92.71 121.16,93.47 113.03,93.47 | IC13.12 113.03,93.47 | v92.96,95 v90.68,97.28 | 113.03,93.47 v113.03,94.49
  Bottom 0.305: v90.68,97.28 v69.09,97.28 | v92.96,95 93.73,94.23 105.41,94.23 105.66,94.49 v113.03,94.49
T100  (via drill 0.61)
  Top 0.305: 107.95,66.04 106.17,67.82 v106.17,93.47 | 107.95,66.04 IC12.2 | X1.7 96.01,10.92 96.01,14.22 100.33,18.54 100.33,58.42 107.95,66.04
  Bottom 0.305: IC1.14 19.81,93.47 v106.17,93.47 136.4,93.47 IC14.11
T101  (via drill 0.61)
  Top 0.305: IC12.1 v107.95,60.45 109.22,59.18 109.22,36.83 104.9,32.51 104.9,4.06 v105.16,3.81 | v25.15,96.27 IC1.13 | v73.91,96.27 77.47,92.71 77.47,88.9 80.52,85.85 v80.52,65.02 | v96.52,3.81 X1.8
  Bottom 0.305: v107.95,60.45 107.7,60.71 89.15,60.71 IC10.1 82.04,63.5 v80.52,65.02 | v73.91,96.27 v25.15,96.27 | v105.16,3.81 v96.52,3.81
T_SR  (via drill 0.61)
  Top 0.305: IC9.6 97.79,24.13 97.79,57.15 104.39,63.75 104.39,65.79 100.33,69.85 100.33,80.26 101.85,81.79 102.87,81.79 v102.87,96.27 | IC11.10 96.52,94.49 v98.04,96.01 98.04,98.55 74.68,98.55 72.39,96.27 72.39,90.17 69.85,87.63 69.85,82.55 66.04,78.74 66.04,69.85 63.5,67.31 63.5,62.23 61.72,60.45 61.72,40.64 v63.75,38.61 | IC18.13 67.82,32.26 67.82,35.05 68.33,35.56 68.33,36.58 v66.04,38.86 | v128.78,96.01 IC14.13
  Bottom 0.305: v98.04,96.01 98.3,96.27 v102.87,96.27 103.12,96.01 104.65,96.01 104.9,96.27 113.79,96.27 114.05,96.01 v128.78,96.01 | v66.04,38.86 65.79,38.61 v63.75,38.61
TA_CLK  (via drill 0.61)
  Top 0.305: R7.1 R8.2 | v65.79,4.06 X1.32 | v94.74,3.81 95.76,2.79 104.14,2.79 104.14,33.27 v104.39,33.53
  Bottom 0.305: v65.79,4.06 66.04,4.32 92.46,4.32 92.96,3.81 v94.74,3.81 | v104.39,33.53 104.65,33.27 134.37,33.27 R7.1
TA_CLR  (via drill 0.61)
  Top 0.305: R5.1 R6.2 | X1.31 63.5,12.95 v66.55,16
  Bottom 0.305: v66.55,16 66.8,16.26 70.1,16.26 70.36,16 74.93,16 75.44,16.51 98.04,16.51 99.57,18.03 118.36,18.03 119.38,19.05 131.57,19.05 134.11,21.59 138.43,21.59 R6.2
TA_J  (via drill 0.61)
  Top 0.305: R2.1 R4.2 | v66.04,12.45 X1.29
  Bottom 0.305: v66.04,12.45 66.29,12.19 77.98,12.19 78.99,13.21 130.05,13.21 130.3,12.95 132.33,12.95 137.16,17.78 R4.2
TA_M
  Top 0.305: R9.1 R10.2
  Bottom 0.305: X1.28 69.85,7.62 74.17,7.62 74.93,8.38 74.93,11.43 78.23,11.43 78.99,12.19 96.27,12.19 97.28,11.18 105.16,11.18 105.41,11.43 145.29,11.43 152.65,18.8 152.65,20.32 R10.2
TA_T  (via drill 0.61)
  Top 0.305: v130.81,13.97 R3.1 | X1.27 v68.58,13.21 68.58,14.48 66.55,14.48 v64.52,12.45 | IC2.10 51.31,93.47 41.91,93.47 41.91,90.17 33.02,81.28 33.02,22.61 v43.18,12.45
  Bottom 0.305: v130.81,13.97 72.64,13.97 71.88,13.21 v68.58,13.21 | v64.52,12.45 v43.18,12.45
TA_W
  Top 0.305: IC8.10 53.85,29.97 53.85,28.96 54.61,28.19 54.61,10.92 57.91,7.62 66.04,7.62 X1.30 66.04,6.1 66.8,5.33 66.8,2.29 83.06,2.29 83.57,2.79 83.57,3.3 85.6,3.3 86.11,2.79 86.11,1.52 140.46,1.52 143.51,4.57 143.51,11.43 141.48,11.43 133.35,19.56 133.35,24.13 R1.1
W0  (via drill 0.61)
  Top 0.305: v69.6,33.53 71.12,32 IC18.11 74.93,26.67 74.93,16.51 v75.95,15.49 | X1.22 74.93,5.08 72.64,5.08 72.64,5.59 72.39,5.84 72.39,6.86 71.63,7.62 69.85,7.62 69.85,13.21 69.6,13.46 69.6,14.99 v69.34,15.24
  Bottom 0.305: IC8.14 45.97,33.27 69.34,33.27 v69.6,33.53 | v69.34,15.24 75.69,15.24 v75.95,15.49
W1  (via drill 0.61)
  Top 0.305: v52.83,11.43 46.99,17.27 46.99,29.21 IC8.13 45.72,32.77 v47.24,34.29 | IC18.10 71.12,33.02 v71.12,33.53
  Bottom 0.305: v52.83,11.43 54.1,10.16 72.39,10.16 X1.23 | v71.12,33.53 70.1,34.54 68.33,34.54 67.82,34.04 47.5,34.04 v47.24,34.29
W2  (via drill 0.61)
  Top 0.305: IC8.12 48.51,30.23 48.51,25.15 49.02,24.64 | 49.02,24.64 49.53,24.13 v49.53,16.76 | v71.37,14.22 72.39,13.21 72.39,7.87 73.66,6.6 X1.24 | IC18.9 76.71,30.99 76.71,40.64 v76.96,40.89 | v53.59,37.85 52.07,36.32 52.07,27.69 49.02,24.64
  Bottom 0.305: v49.53,16.76 51.82,14.48 68.58,14.48 68.83,14.22 v71.37,14.22 | v76.96,40.89 76.71,41.15 58.42,41.15 55.12,37.85 v53.59,37.85
W_SR  (via drill 0.61)
  Top 0.305: IC19.3 67.82,64.01 67.82,69.09 68.58,69.85 v68.58,76.45 | v47.24,77.47 46.99,77.22 46.99,54.61 44.45,52.07 44.45,46.99 46.99,44.45 v46.99,40.13 | v64.77,36.58 67.31,36.58 v67.31,36.07 | v78.49,36.32 78.74,36.07 IC18.8
  Bottom 0.305: v68.58,76.45 67.56,77.47 v47.24,77.47 | v46.99,40.13 50.29,36.83 57.15,36.83 57.4,37.08 62.74,37.08 63.25,36.58 v64.77,36.58 | v67.31,36.07 67.56,36.32 v78.49,36.32

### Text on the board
Top: Datumszähler 2000-2099
Bottom: Datumszähler 2000-2099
